PROGRAM IOMapping
VAR
	GasAnalogRead	: ARRAY[250..269] OF AnalogConverter ;
	ExhAnalogRead	: ARRAY[300..335] OF AnalogConverter ;
	OpAnalogRead	: ARRAY[600..607] OF AnalogConverter ;
	AV				: ARRAY[1..250] OF Valve ;
	bEMOStatus		: BOOL;
	aForceOpValve	: ARRAY[1..250] OF BOOL;
	AV65Open: Valve;
	bForceAV65Open: BOOL;
	AV65Close: Valve;
	bForceAV65Close: BOOL;
	AV202Open: Valve;
	AV202Close:Valve ;
	bForceAV202Open: BOOL;
	bForceAV202Close: BOOL;
	AV79Open: Valve;
	bForceAV79Open: BOOL;
	bForceAV79Close: BOOL;
	AV79Close: Valve;
	rO2Range: REAL;
	AV91Open: Valve;
	bForceAV91Open: BOOL;
	AV91Close: Valve;
	bForceAV91Close: BOOL;
END_VAR

Input();
Output();
Analog();
ValveCtrl();
ValveMapping();
PLC_to_PMC();
PMC_to_PLC();

ACTION Analog:
//模拟量读值转换实际读值程序
GasAnalogRead[250](	// PG/PS3 NH3 in pipe pressure
	AnalogRdValue_In_Int:= stGBI.IW250 , 
	AnalogResMin_In_Int:= 0 , 
	AnalogResMax_In_Int:= 32767 , 
	AnalogPhyMin_In_Real:= -0.1 , 
	AnalogPhyMax_In_Real:= 1 , 
	AnalogRdOffset_In_Real:= , 
	ActRdValue_Out_Real=> GVL.stPLCtoPMC.PG3_Pressure );
	
GasAnalogRead[251](	// PG/PS4 NH3-2 in pipe pressure
	AnalogRdValue_In_Int:= stGBI.IW251 , 
	AnalogResMin_In_Int:= 0 , 
	AnalogResMax_In_Int:= 32767 , 
	AnalogPhyMin_In_Real:= -0.1 , 
	AnalogPhyMax_In_Real:= 1 , 
	AnalogRdOffset_In_Real:= , 
	ActRdValue_Out_Real=> GVL.stPLCtoPMC.PG4_Pressure );

GasAnalogRead[252](	// PG/PS5 SiH4 in pipe pressure
	AnalogRdValue_In_Int:= stGBI.IW252 , 
	AnalogResMin_In_Int:= 0 , 
	AnalogResMax_In_Int:= 32767 , 
	AnalogPhyMin_In_Real:= -0.1 , 
	AnalogPhyMax_In_Real:= 1 , 
	AnalogRdOffset_In_Real:= , 
	ActRdValue_Out_Real=> GVL.stPLCtoPMC.PG5_Pressure );

GasAnalogRead[253](	// PG/PS6 N2-2 in pipe pressure
	AnalogRdValue_In_Int:= stGBI.IW253 , 
	AnalogResMin_In_Int:= 0 , 
	AnalogResMax_In_Int:= 32767 , 
	AnalogPhyMin_In_Real:= -0.1 , 
	AnalogPhyMax_In_Real:= 1 , 
	AnalogRdOffset_In_Real:= , 
	ActRdValue_Out_Real=> GVL.stPLCtoPMC.PG6_Pressure );
	
GasAnalogRead[254](	// PG/PS7 NF3 in pipe pressure
	AnalogRdValue_In_Int:= stGBI.IW254 , 
	AnalogResMin_In_Int:= 0 , 
	AnalogResMax_In_Int:= 32767 , 
	AnalogPhyMin_In_Real:= -0.1 , 
	AnalogPhyMax_In_Real:= 1 , 
	AnalogRdOffset_In_Real:= , 
	ActRdValue_Out_Real=> GVL.stPLCtoPMC.PG7_Pressure );
	
GasAnalogRead[255](	// PG/PS8 20%F2/N2 in pipe pressure
	AnalogRdValue_In_Int:= stGBI.IW255 ,  
	AnalogResMin_In_Int:= 0 , 
	AnalogResMax_In_Int:= 32767 , 
	AnalogPhyMin_In_Real:= -0.1 , 
	AnalogPhyMax_In_Real:= 1 , 
	AnalogRdOffset_In_Real:= , 
	ActRdValue_Out_Real=> GVL.stPLCtoPMC.PG8_Pressure );
	
GasAnalogRead[256](	// PG/PS31 N2-10 in pipe pressure
	AnalogRdValue_In_Int:= stGBI.IW256 , 
	AnalogResMin_In_Int:= 0 , 
	AnalogResMax_In_Int:= 32767 , 
	AnalogPhyMin_In_Real:= -0.1 , 
	AnalogPhyMax_In_Real:= 1 , 
	AnalogRdOffset_In_Real:= , 
	ActRdValue_Out_Real=> GVL.stPLCtoPMC.PG31_Pressure );
	
GasAnalogRead[257](	// PG/PS32 N2-11 in pipe pressure
	AnalogRdValue_In_Int:= stGBI.IW257 , 
	AnalogResMin_In_Int:= 0 , 
	AnalogResMax_In_Int:= 32767 , 
	AnalogPhyMin_In_Real:= -0.1 , 
	AnalogPhyMax_In_Real:= 1 , 
	AnalogRdOffset_In_Real:= , 
	ActRdValue_Out_Real=> GVL.stPLCtoPMC.PG32_Pressure );
	
GasAnalogRead[258](	// VG31 tank-1 backward pipe pressure (0~100torr)
	AnalogRdValue_In_Int:= stGBI.IW258 , 
	AnalogResMin_In_Int:= 0 , 
	AnalogResMax_In_Int:= 32767 , 
	AnalogPhyMin_In_Real:= 0 , 
	AnalogPhyMax_In_Real:= 100 , 
	AnalogRdOffset_In_Real:= , 
	ActRdValue_Out_Real=> GVL.stPLCtoPMC.VG31_Pressure );
	
GasAnalogRead[259](	// PG/PS2 HCL pressure
	AnalogRdValue_In_Int:= stGBI.IW259 , 
	AnalogResMin_In_Int:= 0 , 
	AnalogResMax_In_Int:= 32767 , 
	AnalogPhyMin_In_Real:= -0.1 , 
	AnalogPhyMax_In_Real:= 1 , 
	AnalogRdOffset_In_Real:= , 
	ActRdValue_Out_Real=> GVL.stPLCtoPMC.OX_Value );
	
GasAnalogRead[260](	// PS11 N2-8 in pipe pressure
	AnalogRdValue_In_Int:= stGBI.IW260 , 
	AnalogResMin_In_Int:= 1996 , 
	AnalogResMax_In_Int:= 16383 , 
	AnalogPhyMin_In_Real:= 0 , 
	AnalogPhyMax_In_Real:= 1 , 
	AnalogRdOffset_In_Real:= , 
	ActRdValue_Out_Real=> GVL.stPLCtoPMC.PS11_Pressure );
	
GasAnalogRead[261](	// PG/PS1 N2-1 in pipe pressure
	AnalogRdValue_In_Int:= stGBI.IW261 , 
	AnalogResMin_In_Int:= 0 , 
	AnalogResMax_In_Int:= 32767 , 
	AnalogPhyMin_In_Real:= -0.1 , 
	AnalogPhyMax_In_Real:= 1 , 
	AnalogRdOffset_In_Real:= , 
	ActRdValue_Out_Real=> GVL.stPLCtoPMC.PG1_Pressure );
	
GasAnalogRead[262](	// MS2 gas box(左) exhaust pressure
	AnalogRdValue_In_Int:= stGBI.IW262 , 
	AnalogResMin_In_Int:= 0 , 
	AnalogResMax_In_Int:= 32767 , 
	AnalogPhyMin_In_Real:= 0 , 
	AnalogPhyMax_In_Real:= 200 , 
	AnalogRdOffset_In_Real:= , 
	ActRdValue_Out_Real=> GVL.stPLCtoPMC.MS2_Gasboxleft );
	
GasAnalogRead[263]( // MS5 loading area exhaust pressure
	AnalogRdValue_In_Int:= stGBI.IW263 , 
	AnalogResMin_In_Int:= 0 , 
	AnalogResMax_In_Int:= 32767 , 
	AnalogPhyMin_In_Real:= 0 , 
	AnalogPhyMax_In_Real:= 200 , 
	AnalogRdOffset_In_Real:= , 
	ActRdValue_Out_Real=> GVL.stPLCtoPMC.MS5_Loadingarea );
	

//O2 Range judgment
IF NOT stGBI.I201_13 AND stGBI.I201_14 AND stGBI.I201_15 THEN
	rO2Range := 1000000 ; // O2 range 0~100%
END_IF

IF stGBI.I201_13 AND NOT stGBI.I201_14 AND stGBI.I201_15 THEN
	rO2Range := 100000 ; // O2 range 0~10%
END_IF

IF NOT stGBI.I201_13 AND NOT stGBI.I201_14 AND stGBI.I201_15 THEN
	rO2Range := 10000 ; // O2 range 0~1%
END_IF

IF stGBI.I201_13 AND stGBI.I201_14 AND NOT stGBI.I201_15 THEN
	rO2Range := 1000 ; // O2 range 0~1000ppm
END_IF

IF NOT stGBI.I201_13 AND stGBI.I201_14 AND NOT stGBI.I201_15 THEN
	rO2Range := 100 ; // O2 range 0~100ppm
END_IF

IF stGBI.I201_13 AND NOT stGBI.I201_14 AND NOT stGBI.I201_15 THEN
	rO2Range := 10 ; // O2 range 0~10ppm
END_IF

GasAnalogRead[264](	// O2 concention
	AnalogRdValue_In_Int:= stGBI.IW264 ,  
	AnalogResMin_In_Int:= 0 , 
	AnalogResMax_In_Int:= 32767 , 
	AnalogPhyMin_In_Real:= 0 , 
	AnalogPhyMax_In_Real:= rO2Range , 
	AnalogRdOffset_In_Real:= , 
	ActRdValue_Out_Real=> GVL.stPLCtoPMC.OX_Value );
	
GasAnalogRead[265](	// spare
	AnalogRdValue_In_Int:= stGBI.IW265 , 
	AnalogResMin_In_Int:= 0 , 
	AnalogResMax_In_Int:= 32767 , 
	AnalogPhyMin_In_Real:= 0 , 
	AnalogPhyMax_In_Real:= 1 , 
	AnalogRdOffset_In_Real:= , 
	ActRdValue_Out_Real=> );
	
GasAnalogRead[266](	// PG/PS21 Tank-1 forward pipe pressure
	AnalogRdValue_In_Int:= stGBI.IW266 , 
	AnalogResMin_In_Int:= 3277 , 
	AnalogResMax_In_Int:= 16383 , 
	AnalogPhyMin_In_Real:= -100 , 
	AnalogPhyMax_In_Real:= 300 , 
	AnalogRdOffset_In_Real:= , 
	ActRdValue_Out_Real=> GVL.stPLCtoPMC.PG21_Pressure );
	
GasAnalogRead[267](	// PG/PS22 Tank-2 forward pipe pressure
	AnalogRdValue_In_Int:= stGBI.IW267 , 
	AnalogResMin_In_Int:= 3277 , 
	AnalogResMax_In_Int:= 16383 , 
	AnalogPhyMin_In_Real:= -100 , 
	AnalogPhyMax_In_Real:= 300 , 
	AnalogRdOffset_In_Real:= , 
	ActRdValue_Out_Real=> GVL.stPLCtoPMC.PG22_Pressure );
	
GasAnalogRead[268](	// PG/PS23 Tank-3 forward pipe pressure
	AnalogRdValue_In_Int:= stGBI.IW268 , 
	AnalogResMin_In_Int:= 3277 , 
	AnalogResMax_In_Int:= 16383 , 
	AnalogPhyMin_In_Real:= -100 , 
	AnalogPhyMax_In_Real:= 300 , 
	AnalogRdOffset_In_Real:= , 
	ActRdValue_Out_Real=> GVL.stPLCtoPMC.PG23_Pressure );
	
GasAnalogRead[269](	// PS33  LSC tank pressure
	AnalogRdValue_In_Int:= stGBI.IW269 ,  
	AnalogResMin_In_Int:= 3277 , 
	AnalogResMax_In_Int:= 16383 , 
	AnalogPhyMin_In_Real:= -100 , 
	AnalogPhyMax_In_Real:= 500 , 
	AnalogRdOffset_In_Real:= , 
	ActRdValue_Out_Real=> GVL.stPLCtoPMC.PS33_Pressure );	
	
ExhAnalogRead[300](	// FS105 RHC cooling water flow
	AnalogRdValue_In_Int:= stEXHI.IW300 , 
	AnalogResMin_In_Int:= 0 ,
	AnalogResMax_In_Int:= 32767 , 
	AnalogPhyMin_In_Real:= 0 , 
	AnalogPhyMax_In_Real:= 40 , 
	AnalogRdOffset_In_Real:= , 
	ActRdValue_Out_Real=> GVL.stPLCtoPMC.FS105_Flow );
	
ExhAnalogRead[301](	// FS106 Heater jacket cooling water flow
	AnalogRdValue_In_Int:= stEXHI.IW301 , 
	AnalogResMin_In_Int:= 0 ,
	AnalogResMax_In_Int:= 32767 , 
	AnalogPhyMin_In_Real:= 0 , 
	AnalogPhyMax_In_Real:= 16 , 
	AnalogRdOffset_In_Real:= , 
	ActRdValue_Out_Real=> GVL.stPLCtoPMC.FS106_Flow );
	
ExhAnalogRead[302](	// FS202 Furnace cooling water flow
	AnalogRdValue_In_Int:= stEXHI.IW302 , 
	AnalogResMin_In_Int:= 0 ,
	AnalogResMax_In_Int:= 32767 , 
	AnalogPhyMin_In_Real:= 0 , 
	AnalogPhyMax_In_Real:= 16 , 
	AnalogRdOffset_In_Real:= , 
	ActRdValue_Out_Real=> GVL.stPLCtoPMC.FS202_Flow );
	
ExhAnalogRead[303](	// FS104 Shutter cooling water flow
	AnalogRdValue_In_Int:= stEXHI.IW303 , 
	AnalogResMin_In_Int:= 0 ,
	AnalogResMax_In_Int:= 32767 , 
	AnalogPhyMin_In_Real:= 0 , 
	AnalogPhyMax_In_Real:= 4 , 
	AnalogRdOffset_In_Real:= , 
	ActRdValue_Out_Real=> GVL.stPLCtoPMC.FS104_Flow );
	
ExhAnalogRead[304](	// FS111 boat rotation cooling water flow
	AnalogRdValue_In_Int:= stEXHI.IW304 , 
	AnalogResMin_In_Int:= 0 ,
	AnalogResMax_In_Int:= 32767 , 
	AnalogPhyMin_In_Real:= 0 , 
	AnalogPhyMax_In_Real:= 4 , 
	AnalogRdOffset_In_Real:= , 
	ActRdValue_Out_Real=> GVL.stPLCtoPMC.FS111_Flow );
	
ExhAnalogRead[305](	// FS102 Flange cooling water flow
	AnalogRdValue_In_Int:= stEXHI.IW305 , 
	AnalogResMin_In_Int:= 0 ,
	AnalogResMax_In_Int:= 32767 , 
	AnalogPhyMin_In_Real:= 0 , 
	AnalogPhyMax_In_Real:= 4 , 
	AnalogRdOffset_In_Real:= , 
	ActRdValue_Out_Real=> GVL.stPLCtoPMC.FS102_Flow );
	
ExhAnalogRead[306](	// spare
	AnalogRdValue_In_Int:= stEXHI.IW306 , 
	AnalogResMin_In_Int:= 0 ,
	AnalogResMax_In_Int:= 32767 , 
	AnalogPhyMin_In_Real:= 0 , 
	AnalogPhyMax_In_Real:= 1 , 
	AnalogRdOffset_In_Real:= , 
	ActRdValue_Out_Real=> );
	
ExhAnalogRead[307](	// spare
	AnalogRdValue_In_Int:= stEXHI.IW307 , 
	AnalogResMin_In_Int:= 0 ,
	AnalogResMax_In_Int:= 32767 , 
	AnalogPhyMin_In_Real:= 0 , 
	AnalogPhyMax_In_Real:= 1 , 
	AnalogRdOffset_In_Real:= , 
	ActRdValue_Out_Real=> );
	
ExhAnalogRead[308](	// DG1 tube and loading area differential pressure
	AnalogRdValue_In_Int:= stEXHI.IW308 , 
	AnalogResMin_In_Int:= 0 ,
	AnalogResMax_In_Int:= 32767 , 
	AnalogPhyMin_In_Real:= -300 , 
	AnalogPhyMax_In_Real:= 300 , 
	AnalogRdOffset_In_Real:= , 
	ActRdValue_Out_Real=> GVL.stPLCtoPMC.DG1_Pressure );
	
ExhAnalogRead[309](	// spare
	AnalogRdValue_In_Int:= stEXHI.IW309 , 
	AnalogResMin_In_Int:= 0 ,
	AnalogResMax_In_Int:= 32767 , 
	AnalogPhyMin_In_Real:= 0 , 
	AnalogPhyMax_In_Real:= 1 , 
	AnalogRdOffset_In_Real:= , 
	ActRdValue_Out_Real=> );
	
ExhAnalogRead[310](	// spare
	AnalogRdValue_In_Int:= stEXHI.IW310 , 
	AnalogResMin_In_Int:= 0 ,
	AnalogResMax_In_Int:= 32767 , 
	AnalogPhyMin_In_Real:= 0 , 
	AnalogPhyMax_In_Real:= 1 , 
	AnalogRdOffset_In_Real:= , 
	ActRdValue_Out_Real=> );
	
ExhAnalogRead[311](	// FS116 Cooling unit flow
	AnalogRdValue_In_Int:= stEXHI.IW311 , 
	AnalogResMin_In_Int:= 0 ,
	AnalogResMax_In_Int:= 32767 , 
	AnalogPhyMin_In_Real:= 0 , 
	AnalogPhyMax_In_Real:= 16 , 
	AnalogRdOffset_In_Real:= , 
	ActRdValue_Out_Real=> GVL.stPLCtoPMC.FS116_Flow );
	
ExhAnalogRead[312](	// PS13 pressure
	AnalogRdValue_In_Int:= stEXHI.IW312 , 
	AnalogResMin_In_Int:= 0 ,
	AnalogResMax_In_Int:= 32767 , 
	AnalogPhyMin_In_Real:= 0 , 
	AnalogPhyMax_In_Real:= 98.1 , 
	AnalogRdOffset_In_Real:= , 
	ActRdValue_Out_Real=> GVL.stPLCtoPMC.PS13_Pressure );
	
ExhAnalogRead[313](	// spare
	AnalogRdValue_In_Int:= stEXHI.IW313 , 
	AnalogResMin_In_Int:= 0 ,
	AnalogResMax_In_Int:= 32767 , 
	AnalogPhyMin_In_Real:= 0 , 
	AnalogPhyMax_In_Real:= 1 , 
	AnalogRdOffset_In_Real:= , 
	ActRdValue_Out_Real=> );
	
ExhAnalogRead[314](	// spare
	AnalogRdValue_In_Int:= stEXHI.IW314 , 
	AnalogResMin_In_Int:= 0 ,
	AnalogResMax_In_Int:= 32767 , 
	AnalogPhyMin_In_Real:= 0 , 
	AnalogPhyMax_In_Real:= 1 , 
	AnalogRdOffset_In_Real:= , 
	ActRdValue_Out_Real=> );
	
ExhAnalogRead[315](	// spare
	AnalogRdValue_In_Int:= stEXHI.IW315 , 
	AnalogResMin_In_Int:= 0 ,
	AnalogResMax_In_Int:= 32767 , 
	AnalogPhyMin_In_Real:= 0 , 
	AnalogPhyMax_In_Real:= 1 , 
	AnalogRdOffset_In_Real:= , 
	ActRdValue_Out_Real=> );
	
ExhAnalogRead[316](	// spare
	AnalogRdValue_In_Int:= stEXHI.IW316 , 
	AnalogResMin_In_Int:= 0 ,
	AnalogResMax_In_Int:= 32767 , 
	AnalogPhyMin_In_Real:= 0 , 
	AnalogPhyMax_In_Real:= 1 , 
	AnalogRdOffset_In_Real:= , 
	ActRdValue_Out_Real=> );
	
ExhAnalogRead[317](	// spare
	AnalogRdValue_In_Int:= stEXHI.IW317 , 
	AnalogResMin_In_Int:= 0 ,
	AnalogResMax_In_Int:= 32767 , 
	AnalogPhyMin_In_Real:= 0 , 
	AnalogPhyMax_In_Real:= 1 , 
	AnalogRdOffset_In_Real:= , 
	ActRdValue_Out_Real=> );
	
ExhAnalogRead[318](	// PS21 N2-13 in pipe pressure 0.6~5V
	AnalogRdValue_In_Int:= stEXHI.IW318 , 
	AnalogResMin_In_Int:= 3276 ,
	AnalogResMax_In_Int:= 16383 , 
	AnalogPhyMin_In_Real:= -0.1 , 
	AnalogPhyMax_In_Real:= 1 , 
	AnalogRdOffset_In_Real:= , 
	ActRdValue_Out_Real=> GVL.stPLCtoPMC.PS21_Pressure );
	
ExhAnalogRead[319](	// PS110 exhaust pressure
	AnalogRdValue_In_Int:= stEXHI.IW319 , 
	AnalogResMin_In_Int:= 3276 ,
	AnalogResMax_In_Int:= 16383 , 
	AnalogPhyMin_In_Real:= -100 , 
	AnalogPhyMax_In_Real:= 100 , 
	AnalogRdOffset_In_Real:= , 
	ActRdValue_Out_Real=> GVL.stPLCtoPMC.PS110_Pressure );
	
ExhAnalogRead[320](	// PG/PS12 N2-9 in pipe pressure
	AnalogRdValue_In_Int:= stEXHI.IW320 , 
	AnalogResMin_In_Int:= 0 ,
	AnalogResMax_In_Int:= 32767 , 
	AnalogPhyMin_In_Real:= -0.1 , 
	AnalogPhyMax_In_Real:= 1 , 
	AnalogRdOffset_In_Real:= , 
	ActRdValue_Out_Real=> GVL.stPLCtoPMC.PG12_Pressure );
	
ExhAnalogRead[321](	// VG14 pressure
	AnalogRdValue_In_Int:= stEXHI.IW321 , 
	AnalogResMin_In_Int:= 0 ,
	AnalogResMax_In_Int:= 32767 , 
	AnalogPhyMin_In_Real:= 0 , 
	AnalogPhyMax_In_Real:= 10 , 
	AnalogRdOffset_In_Real:= , 
	ActRdValue_Out_Real=> GVL.stPLCtoPMC.VG14_Pressure );
	
ExhAnalogRead[322](	// PS14 pressure
	AnalogRdValue_In_Int:= stEXHI.IW322 , 
	AnalogResMin_In_Int:= 3276 ,
	AnalogResMax_In_Int:= 16383 , 
	AnalogPhyMin_In_Real:= -100 , 
	AnalogPhyMax_In_Real:= 100 , 
	AnalogRdOffset_In_Real:= , 
	ActRdValue_Out_Real=> GVL.stPLCtoPMC.PS14_Pressure );
	
ExhAnalogRead[323](	// spare
	AnalogRdValue_In_Int:= stEXHI.IW323 , 
	AnalogResMin_In_Int:= 0 ,
	AnalogResMax_In_Int:= 32767 , 
	AnalogPhyMin_In_Real:= 0 , 
	AnalogPhyMax_In_Real:= 1 , 
	AnalogRdOffset_In_Real:= , 
	ActRdValue_Out_Real=> );
	
ExhAnalogRead[324](	// spare
	AnalogRdValue_In_Int:= stEXHI.IW324 , 
	AnalogResMin_In_Int:= 0 ,
	AnalogResMax_In_Int:= 32767 , 
	AnalogPhyMin_In_Real:= 0 , 
	AnalogPhyMax_In_Real:= 1 , 
	AnalogRdOffset_In_Real:= , 
	ActRdValue_Out_Real=> );
	
ExhAnalogRead[325](	// spare
	AnalogRdValue_In_Int:= stEXHI.IW325 , 
	AnalogResMin_In_Int:= 0 ,
	AnalogResMax_In_Int:= 32767 , 
	AnalogPhyMin_In_Real:= 0 , 
	AnalogPhyMax_In_Real:= 1 , 
	AnalogRdOffset_In_Real:= , 
	ActRdValue_Out_Real=> );
	
ExhAnalogRead[326](	// spare
	AnalogRdValue_In_Int:= stEXHI.IW326 , 
	AnalogResMin_In_Int:= 0 ,
	AnalogResMax_In_Int:= 32767 , 
	AnalogPhyMin_In_Real:= 0 , 
	AnalogPhyMax_In_Real:= 1 , 
	AnalogRdOffset_In_Real:= , 
	ActRdValue_Out_Real=> );
	
ExhAnalogRead[327](	// spare
	AnalogRdValue_In_Int:= stEXHI.IW327 , 
	AnalogResMin_In_Int:= 0 ,
	AnalogResMax_In_Int:= 32767 , 
	AnalogPhyMin_In_Real:= 0 , 
	AnalogPhyMax_In_Real:= 1 , 
	AnalogRdOffset_In_Real:= , 
	ActRdValue_Out_Real=> );
	
ExhAnalogRead[328](	// spare
	AnalogRdValue_In_Int:= stEXHI.IW328 , 
	AnalogResMin_In_Int:= 0 ,
	AnalogResMax_In_Int:= 32767 , 
	AnalogPhyMin_In_Real:= 0 , 
	AnalogPhyMax_In_Real:= 1 , 
	AnalogRdOffset_In_Real:= , 
	ActRdValue_Out_Real=> );
	
ExhAnalogRead[329](	// spare
	AnalogRdValue_In_Int:= stEXHI.IW329 , 
	AnalogResMin_In_Int:= 0 ,
	AnalogResMax_In_Int:= 32767 , 
	AnalogPhyMin_In_Real:= 0 , 
	AnalogPhyMax_In_Real:= 1 , 
	AnalogRdOffset_In_Real:= , 
	ActRdValue_Out_Real=> );
	
ExhAnalogRead[330](	// spare
	AnalogRdValue_In_Int:= stEXHI.IW330 , 
	AnalogResMin_In_Int:= 0 ,
	AnalogResMax_In_Int:= 32767 , 
	AnalogPhyMin_In_Real:= 0 , 
	AnalogPhyMax_In_Real:= 1 , 
	AnalogRdOffset_In_Real:= , 
	ActRdValue_Out_Real=> );
	
ExhAnalogRead[331](	// spare
	AnalogRdValue_In_Int:= stEXHI.IW331 , 
	AnalogResMin_In_Int:= 0 ,
	AnalogResMax_In_Int:= 32767 , 
	AnalogPhyMin_In_Real:= 0 , 
	AnalogPhyMax_In_Real:= 1 , 
	AnalogRdOffset_In_Real:= , 
	ActRdValue_Out_Real=> );
	
ExhAnalogRead[332](	// spare
	AnalogRdValue_In_Int:= stEXHI.IW332 , 
	AnalogResMin_In_Int:= 0 ,
	AnalogResMax_In_Int:= 32767 , 
	AnalogPhyMin_In_Real:= 0 , 
	AnalogPhyMax_In_Real:= 1 , 
	AnalogRdOffset_In_Real:= , 
	ActRdValue_Out_Real=> );
	
ExhAnalogRead[333](	// spare
	AnalogRdValue_In_Int:= stEXHI.IW333 , 
	AnalogResMin_In_Int:= 0 ,
	AnalogResMax_In_Int:= 32767 , 
	AnalogPhyMin_In_Real:= 0 , 
	AnalogPhyMax_In_Real:= 1 , 
	AnalogRdOffset_In_Real:= , 
	ActRdValue_Out_Real=> );
	
ExhAnalogRead[334](	// spare
	AnalogRdValue_In_Int:= stEXHI.IW334 , 
	AnalogResMin_In_Int:= 0 ,
	AnalogResMax_In_Int:= 32767 , 
	AnalogPhyMin_In_Real:= 0 , 
	AnalogPhyMax_In_Real:= 1 , 
	AnalogRdOffset_In_Real:= , 
	ActRdValue_Out_Real=> );
	
ExhAnalogRead[335](	// spare
	AnalogRdValue_In_Int:= stEXHI.IW335 , 
	AnalogResMin_In_Int:= 0 ,
	AnalogResMax_In_Int:= 32767 , 
	AnalogPhyMin_In_Real:= 0 , 
	AnalogPhyMax_In_Real:= 1 , 
	AnalogRdOffset_In_Real:= , 
	ActRdValue_Out_Real=> );
	
OpAnalogRead[600](	// MS8 RHC exhaust pressure
	AnalogRdValue_In_Int:= stOPI.IW600 , 
	AnalogResMin_In_Int:= 0 ,
	AnalogResMax_In_Int:= 32767 , 
	AnalogPhyMin_In_Real:= 0 , 
	AnalogPhyMax_In_Real:= 2 , 
	AnalogRdOffset_In_Real:= , 
	ActRdValue_Out_Real=> GVL.stPLCtoPMC.MS8_RHC_ExhPress );
	
OpAnalogRead[601](	// MS1 Heater exhaust pressure
	AnalogRdValue_In_Int:= stOPI.IW601 , 
	AnalogResMin_In_Int:= 0 ,
	AnalogResMax_In_Int:= 32767 , 
	AnalogPhyMin_In_Real:= 0 , 
	AnalogPhyMax_In_Real:= 200 , 
	AnalogRdOffset_In_Real:= , 
	ActRdValue_Out_Real=> GVL.stPLCtoPMC.MS1_Heater );
	
OpAnalogRead[602](	// MS3 Scavenger exhaust pressure
	AnalogRdValue_In_Int:= stOPI.IW602 , 
	AnalogResMin_In_Int:= 0 ,
	AnalogResMax_In_Int:= 32767 , 
	AnalogPhyMin_In_Real:= 0 , 
	AnalogPhyMax_In_Real:= 200 , 
	AnalogRdOffset_In_Real:= , 
	ActRdValue_Out_Real=> GVL.stPLCtoPMC.MS3_Scavenger );
	
OpAnalogRead[603](	// MS6 Frontbody exhaust pressure
	AnalogRdValue_In_Int:= stOPI.IW603 , 
	AnalogResMin_In_Int:= 0 ,
	AnalogResMax_In_Int:= 32767 , 
	AnalogPhyMin_In_Real:= 0 , 
	AnalogPhyMax_In_Real:= 200 , 
	AnalogRdOffset_In_Real:= , 
	ActRdValue_Out_Real=> GVL.stPLCtoPMC.MS6_Frontbody );
	
OpAnalogRead[604](	// MS9 LSC1 exhaust pressure
	AnalogRdValue_In_Int:= stOPI.IW604 , 
	AnalogResMin_In_Int:= 0 ,
	AnalogResMax_In_Int:= 32767 , 
	AnalogPhyMin_In_Real:= 0 , 
	AnalogPhyMax_In_Real:= 200 , 
	AnalogRdOffset_In_Real:= , 
	ActRdValue_Out_Real=> GVL.stPLCtoPMC.MS9_LSC1 );
	
OpAnalogRead[605](	// MS11 Gas box(右上) exhaust pressure
	AnalogRdValue_In_Int:= stOPI.IW605 , 
	AnalogResMin_In_Int:= 0 ,
	AnalogResMax_In_Int:= 32767 , 
	AnalogPhyMin_In_Real:= 0 , 
	AnalogPhyMax_In_Real:= 200 , 
	AnalogRdOffset_In_Real:= , 
	ActRdValue_Out_Real=> GVL.stPLCtoPMC.MS11_GasBox );
	
OpAnalogRead[606](	// MS12 Gas box(右下) exhaust pressure
	AnalogRdValue_In_Int:= stOPI.IW606 , 
	AnalogResMin_In_Int:= 0 ,
	AnalogResMax_In_Int:= 32767 , 
	AnalogPhyMin_In_Real:= 0 , 
	AnalogPhyMax_In_Real:= 200 , 
	AnalogRdOffset_In_Real:= , 
	ActRdValue_Out_Real=> GVL.stPLCtoPMC.MS12_GasBox );
	
OpAnalogRead[607](	// spare
	AnalogRdValue_In_Int:= stOPI.IW607 , 
	AnalogResMin_In_Int:= 0 ,
	AnalogResMax_In_Int:= 32767 , 
	AnalogPhyMin_In_Real:= 0 , 
	AnalogPhyMax_In_Real:= 200 , 
	AnalogRdOffset_In_Real:= , 
	ActRdValue_Out_Real=> );
END_ACTION

ACTION Input:
//************************************************************************
//02.Gas Box INput/OUTPUT(气体柜输入/出映射）
//************************************************************************
stGBI.	I200_00	:=		GB_EL1889[1,0]	;
stGBI.	I200_01	:=		GB_EL1889[1,1]	;
stGBI.	I200_02	:=		GB_EL1889[1,2]	;
stGBI.	I200_03	:=		GB_EL1889[1,3]	;
stGBI.	I200_04	:=		GB_EL1889[1,4]	;
stGBI.	I200_05	:=		GB_EL1889[1,5]	;
stGBI.	I200_06	:=		GB_EL1889[1,6]	;
stGBI.	I200_07	:=		GB_EL1889[1,7]	;
stGBI.	I200_08	:=		GB_EL1889[1,8]	;
stGBI.	I200_09	:=		GB_EL1889[1,9]	;
stGBI.	I200_10	:=		GB_EL1889[1,10]	;
stGBI.	I200_11	:=		GB_EL1889[1,11]	;
stGBI.	I200_12	:=		GB_EL1889[1,12]	;
stGBI.	I200_13	:=		GB_EL1889[1,13]	;
stGBI.	I200_14	:=		GB_EL1889[1,14]	;
stGBI.	I200_15	:=		GB_EL1889[1,15]	;
stGBI.	I201_00	:=		GB_EL1889[2,0]	;
stGBI.	I201_01	:=		GB_EL1889[2,1]	;
stGBI.	I201_02	:=		GB_EL1889[2,2]	;
stGBI.	I201_03	:=		GB_EL1889[2,3]	;
stGBI.	I201_04	:=		GB_EL1889[2,4]	;
stGBI.	I201_05	:=		GB_EL1889[2,5]	;
stGBI.	I201_06	:=		GB_EL1889[2,6]	;
stGBI.	I201_07	:=		GB_EL1889[2,7]	;
stGBI.	I201_08	:=		GB_EL1889[2,8]	;
stGBI.	I201_09	:=		GB_EL1889[2,9]	;
stGBI.	I201_10	:=		GB_EL1889[2,10]	;
stGBI.	I201_11	:=		GB_EL1889[2,11]	;
stGBI.	I201_12	:=		GB_EL1889[2,12]	;
stGBI.	I201_13	:=		GB_EL1889[2,13]	;
stGBI.	I201_14	:=		GB_EL1889[2,14]	;
stGBI.	I201_15	:=		GB_EL1889[2,15]	;
stGBI.	I203_00	:=		GB_EL1889[3,0]	;
stGBI.	I203_01	:=		GB_EL1889[3,1]	;
stGBI.	I203_02	:=		GB_EL1889[3,2]	;
stGBI.	I203_03	:=		GB_EL1889[3,3]	;
stGBI.	I203_04	:=		GB_EL1889[3,4]	;
stGBI.	I203_05	:=		GB_EL1889[3,5]	;
stGBI.	I203_06	:=		GB_EL1889[3,6]	;
stGBI.	I203_07	:=		GB_EL1889[3,7]	;
stGBI.	I203_08	:=		GB_EL1889[3,8]	;
stGBI.	I203_09	:=		GB_EL1889[3,9]	;
stGBI.	I203_10	:=		GB_EL1889[3,10]	;
stGBI.	I203_11	:=		GB_EL1889[3,11]	;
stGBI.	I203_12	:=		GB_EL1889[3,12]	;
stGBI.	I203_13	:=		GB_EL1889[3,13]	;
stGBI.	I203_14	:=		GB_EL1889[3,14]	;
stGBI.	I203_15	:=		GB_EL1889[3,15]	;

stGBI.	IW250	:=		GB_EL3164[1,	1]	;
stGBI.	IW251	:=		GB_EL3164[1,	2]	;
stGBI.	IW252	:=		GB_EL3164[1,	3]	;
stGBI.	IW253	:=		GB_EL3164[1,	4]	;
stGBI.	IW254	:=		GB_EL3164[2,	1]	;
stGBI.	IW255	:=		GB_EL3164[2,	2]	;
stGBI.	IW256	:=		GB_EL3164[2,	3]	;
stGBI.	IW257	:=		GB_EL3164[2,	4]	;
stGBI.	IW258	:=		GB_EL3164[3,	1]	;
stGBI.	IW259	:=		GB_EL3164[3,	2]	;
stGBI.	IW260	:=		GB_EL3164[3,	3]	;
stGBI.	IW261	:=		GB_EL3164[3,	4]	;
stGBI.	IW262	:=		GB_EL3124[1,	1]	;
stGBI.	IW263	:=		GB_EL3124[1,	2]	;
stGBI.	IW264	:=		GB_EL3124[1,	3]	;
stGBI.	IW265	:=		GB_EL3124[1,	4]	;
stGBI.	IW266	:=		GB_EL3164[4,	1]	;
stGBI.	IW267	:=		GB_EL3164[4,	2]	;
stGBI.	IW268	:=		GB_EL3164[4,	3]	;
stGBI.	IW269	:=		GB_EL3164[4,	4]	;


//************************************************************************
//03.EXH Box INput/OUTPUT(排气柜输入/出映射）
//************************************************************************
stEXHI.	I300_00	:=		EXH_EL1889[1,0]	;
stEXHI.	I300_01	:=		EXH_EL1889[1,1]	;
stEXHI.	I300_02	:=		EXH_EL1889[1,2]	;
stEXHI.	I300_03	:=		EXH_EL1889[1,3]	;
stEXHI.	I300_04	:=		EXH_EL1889[1,4]	;
stEXHI.	I300_05	:=		EXH_EL1889[1,5]	;
stEXHI.	I300_06	:=		EXH_EL1889[1,6]	;
stEXHI.	I300_07	:=		EXH_EL1889[1,7]	;
stEXHI.	I300_08	:=		EXH_EL1889[1,8]	;
stEXHI.	I300_09	:=		EXH_EL1889[1,9]	;
stEXHI.	I300_10	:=		EXH_EL1889[1,10]	;
stEXHI.	I300_11	:=		EXH_EL1889[1,11]	;
stEXHI.	I300_12	:=		EXH_EL1889[1,12]	;
stEXHI.	I300_13	:=		EXH_EL1889[1,13]	;
stEXHI.	I300_14	:=		EXH_EL1889[1,14]	;
stEXHI.	I300_15	:=		EXH_EL1889[1,15]	;
stEXHI.	I301_00	:=		EXH_EL1889[2,0]	;
stEXHI.	I301_01	:=		EXH_EL1889[2,1]	;
stEXHI.	I301_02	:=		EXH_EL1889[2,2]	;
stEXHI.	I301_03	:=		EXH_EL1889[2,3]	;
stEXHI.	I301_04	:=		EXH_EL1889[2,4]	;
stEXHI.	I301_05	:=		EXH_EL1889[2,5]	;
stEXHI.	I301_06	:=		EXH_EL1889[2,6]	;
stEXHI.	I301_07	:=		EXH_EL1889[2,7]	;
stEXHI.	I301_08	:=		EXH_EL1889[2,8]	;
stEXHI.	I301_09	:=		EXH_EL1889[2,9]	;
stEXHI.	I301_10	:=		EXH_EL1889[2,10]	;
stEXHI.	I301_11	:=		EXH_EL1889[2,11]	;
stEXHI.	I301_12	:=		EXH_EL1889[2,12]	;
stEXHI.	I301_13	:=		EXH_EL1889[2,13]	;
stEXHI.	I301_14	:=		EXH_EL1889[2,14]	;
stEXHI.	I301_15	:=		EXH_EL1889[2,15]	;
stEXHI.	I302_00	:=		EXH_EL1889[3,0]	;
stEXHI.	I302_01	:=		EXH_EL1889[3,1]	;
stEXHI.	I302_02	:=		EXH_EL1889[3,2]	;
stEXHI.	I302_03	:=		EXH_EL1889[3,3]	;
stEXHI.	I302_04	:=		EXH_EL1889[3,4]	;
stEXHI.	I302_05	:=		EXH_EL1889[3,5]	;
stEXHI.	I302_06	:=		EXH_EL1889[3,6]	;
stEXHI.	I302_07	:=		EXH_EL1889[3,7]	;
stEXHI.	I302_08	:=		EXH_EL1889[3,8]	;
stEXHI.	I302_09	:=		EXH_EL1889[3,9]	;
stEXHI.	I302_10	:=		EXH_EL1889[3,10]	;
stEXHI.	I302_11	:=		EXH_EL1889[3,11]	;
stEXHI.	I302_12	:=		EXH_EL1889[3,12]	;
stEXHI.	I302_13	:=		EXH_EL1889[3,13]	;
stEXHI.	I302_14	:=		EXH_EL1889[3,14]	;
stEXHI.	I302_15	:=		EXH_EL1889[3,15]	;
stEXHI.	I303_00	:=		EXH_EL1889[4,0]	;
stEXHI.	I303_01	:=		EXH_EL1889[4,1]	;
stEXHI.	I303_02	:=		EXH_EL1889[4,2]	;
stEXHI.	I303_03	:=		EXH_EL1889[4,3]	;
stEXHI.	I303_04	:=		EXH_EL1889[4,4]	;
stEXHI.	I303_05	:=		EXH_EL1889[4,5]	;
stEXHI.	I303_06	:=		EXH_EL1889[4,6]	;
stEXHI.	I303_07	:=		EXH_EL1889[4,7]	;
stEXHI.	I303_08	:=		EXH_EL1889[4,8]	;
stEXHI.	I303_09	:=		EXH_EL1889[4,9]	;
stEXHI.	I303_10	:=		EXH_EL1889[4,10]	;
stEXHI.	I303_11	:=		EXH_EL1889[4,11]	;
stEXHI.	I303_12	:=		EXH_EL1889[4,12]	;
stEXHI.	I303_13	:=		EXH_EL1889[4,13]	;
stEXHI.	I303_14	:=		EXH_EL1889[4,14]	;
stEXHI.	I303_15	:=		EXH_EL1889[4,15]	;
stEXHI.	I304_00	:=		EXH_EL1889[5,0]	;
stEXHI. I304_01	:=		EXH_EL1889[5,1]	;
stEXHI. I304_02	:=		EXH_EL1889[5,2]	;
stEXHI. I304_03	:=		EXH_EL1889[5,3]	;
stEXHI. I304_04	:=		EXH_EL1889[5,4]	;
stEXHI. I304_05	:=		EXH_EL1889[5,5]	;
stEXHI. I304_06	:=		EXH_EL1889[5,6]	;
stEXHI. I304_07	:=		EXH_EL1889[5,7]	;
stEXHI. I304_08	:=		EXH_EL1889[5,8]	;
stEXHI. I304_09	:=		EXH_EL1889[5,9]	;
stEXHI. I304_10	:=		EXH_EL1889[5,10]	;
stEXHI. I304_11	:=		EXH_EL1889[5,11]	;
stEXHI. I304_12	:=		EXH_EL1889[5,12]	;
stEXHI. I304_13	:=		EXH_EL1889[5,13]	;
stEXHI. I304_14	:=		EXH_EL1889[5,14]	;
stEXHI. I304_15	:=		EXH_EL1889[5,15]	;

stEXHI.	IW300	:=		EXH_EL3124[1,	1]	;
stEXHI.	IW301	:=		EXH_EL3124[1,	2]	;
stEXHI.	IW302	:=		EXH_EL3124[1,	3]	;
stEXHI.	IW303	:=		EXH_EL3124[1,	4]	;
stEXHI.	IW304	:=		EXH_EL3124[2,	1]	;
stEXHI.	IW305	:=		EXH_EL3124[2,	2]	;
stEXHI.	IW306	:=		EXH_EL3124[2,	3]	;
stEXHI.	IW307	:=		EXH_EL3124[2,	4]	;
stEXHI.	IW308	:=		EXH_EL3124[3,	1]	;
stEXHI.	IW309	:=		EXH_EL3124[3,	2]	;
stEXHI.	IW310	:=		EXH_EL3124[3,	3]	;
stEXHI.	IW311	:=		EXH_EL3124[3,	4]	;
stEXHI.	IW312	:=		EXH_EL3124[4,	1]	;
stEXHI.	IW313	:=		EXH_EL3124[4,	2]	;
stEXHI.	IW314	:=		EXH_EL3124[4,	3]	;
stEXHI.	IW315	:=		EXH_EL3124[4,	4]	;
stEXHI.	IW316	:=		EXH_EL3164[1,	1]	;
stEXHI.	IW317	:=		EXH_EL3164[1,	2]	;
stEXHI.	IW318	:=		EXH_EL3164[1,	3]	;
stEXHI.	IW319	:=		EXH_EL3164[1,	4]	;
stEXHI.	IW320	:=		EXH_EL3164[2,	1]	;
stEXHI.	IW321	:=		EXH_EL3164[2,	2]	;
stEXHI.	IW322	:=		EXH_EL3164[2,	3]	;
stEXHI.	IW323	:=		EXH_EL3164[2,	4]	;
stEXHI.	IW324	:=		EXH_EL3164[3,	1]	;
stEXHI.	IW325	:=		EXH_EL3164[3,	2]	;
stEXHI.	IW326	:=		EXH_EL3164[3,	3]	;
stEXHI.	IW327	:=		EXH_EL3164[3,	4]	;
stEXHI.	IW328	:=		EXH_EL3164[4,	1]	;
stEXHI.	IW329	:=		EXH_EL3164[4,	2]	;
stEXHI.	IW330	:=		EXH_EL3164[4,	3]	;
stEXHI.	IW331	:=		EXH_EL3164[4,	4]	;
stEXHI.	IW332	:=		EXH_EL3124[5,	1]	;
stEXHI.	IW333	:=		EXH_EL3124[5,	2]	;
stEXHI.	IW334	:=		EXH_EL3124[5,	3]	;
stEXHI.	IW335	:=		EXH_EL3124[5,	4]	;

//************************************************************************
//06.OP Box INput/OUTPUT(天桥内PLC输入/出映射）
//************************************************************************
stOPI.	I600_00	:=		OP_EL1889[1,0]	;
stOPI.	I600_01	:=		OP_EL1889[1,1]	;
stOPI.	I600_02	:=		OP_EL1889[1,2]	;
stOPI.	I600_03	:=		OP_EL1889[1,3]	;
stOPI.	I600_04	:=		OP_EL1889[1,4]	;
stOPI.	I600_05	:=		OP_EL1889[1,5]	;
stOPI.	I600_06	:=		OP_EL1889[1,6]	;
stOPI.	I600_07	:=		OP_EL1889[1,7]	;
stOPI.	I600_08	:=		OP_EL1889[1,8]	;
stOPI.	I600_09	:=		OP_EL1889[1,9]	;
stOPI.	I600_10	:=		OP_EL1889[1,10]	;
stOPI.	I600_11	:=		OP_EL1889[1,11]	;
stOPI.	I600_12	:=		OP_EL1889[1,12]	;
stOPI.	I600_13	:=		OP_EL1889[1,13]	;
stOPI.	I600_14	:=		OP_EL1889[1,14]	;
stOPI.	I600_15	:=		OP_EL1889[1,15]	;

stOPI.	IW600	:=		OP_EL3124[1,	1]	;
stOPI.	IW601	:=		OP_EL3124[1,	2]	;
stOPI.	IW602	:=		OP_EL3124[1,	3]	;
stOPI.	IW603	:=		OP_EL3124[1,	4]	;
stOPI.	IW604	:=		OP_EL3124[2,	1]	;
stOPI.	IW605	:=		OP_EL3124[2,	2]	;
stOPI.	IW606	:=		OP_EL3124[2,	3]	;
stOPI.	IW607	:=		OP_EL3124[2,	4]	;
END_ACTION

ACTION Output:
//========================================================================
//!!!!!!!!!!!!!!!!!!!!以下依托于硬件，硬件无变动禁止更改!!!!!!!!!!!!!!!!!!
//=======================================================================

//************************************************************************
//02.Gas Box INput/OUTPUT(气体柜输入/出映射）
//************************************************************************
GB_EL2889[1,0]	:=	FALSE(*stGBQ.	Q200_00*)	;
GB_EL2889[1,1]	:=	stGBQ.	Q200_01	;
GB_EL2889[1,2]	:=	stGBQ.	Q200_02	;
GB_EL2889[1,3]	:=	stGBQ.	Q200_03	;
GB_EL2889[1,4]	:=	stGBQ.	Q200_04	;
GB_EL2889[1,5]	:=	stGBQ.	Q200_05	;
GB_EL2889[1,6]	:=	stGBQ.	Q200_06	;
GB_EL2889[1,7]	:=	stGBQ.	Q200_07	;
GB_EL2889[1,8]	:=	stGBQ.	Q200_08	;
GB_EL2889[1,9]	:=	stGBQ.	Q200_09	;
GB_EL2889[1,10]	:=	stGBQ.	Q200_10	;
GB_EL2889[1,11]	:=	stGBQ.	Q200_11	;
GB_EL2889[1,12]	:=	stGBQ.	Q200_12	;
GB_EL2889[1,13]	:=	stGBQ.	Q200_13	;
GB_EL2889[1,14]	:=	stGBQ.	Q200_14	;
GB_EL2889[1,15]	:=	stGBQ.	Q200_15	;

GB_EV := stGBQ.QEV ;

//************************************************************************
//03.EXH Box INput/OUTPUT(排气柜输入/出映射）
//************************************************************************
EXH_EL2889[1,0]		:=	NOT GVL.stPMCtoPLC.WAT_R_sw OR ( GVL.stPMCtoPLC.R_Axis_Temp > 80 ) (*stEXHQ.	Q300_00*)	;
EXH_EL2889[1,1]		:=	FALSE(*NOT GVL.stPMCtoPLC.WAT_F_sw OR 
						(	
							( GVL.stPMCtoPLC.Inlet_Ht_1_temp > 200) OR 
							( GVL.stPMCtoPLC.Inlet_Ht_2_temp > 200) OR
							( GVL.stPMCtoPLC.Port_Ht_1_temp > 200) 	OR
							( GVL.stPMCtoPLC.Port_Ht_2_temp > 200) 	OR
							( GVL.stPMCtoPLC.Port_Ht_3_temp > 200) 	OR
							( GVL.stPMCtoPLC.Port_Ht_4_temp > 200) 	OR
							( GVL.stPMCtoPLC.Port_Ht_5_temp > 200) 	
						)*)(*stEXHQ.	Q300_01*)	;
EXH_EL2889[1,2]		:=	stEXHQ.	Q300_02	;
EXH_EL2889[1,3]		:=	stEXHQ.	Q300_03	;
EXH_EL2889[1,4]		:=	stEXHQ.	Q300_04	;
EXH_EL2889[1,5]		:=	stEXHQ.	Q300_05	;
EXH_EL2889[1,6]		:=	stEXHQ.	Q300_06	;
EXH_EL2889[1,7]		:=	stEXHQ.	Q300_07	;
EXH_EL2889[1,8]		:=	TRUE(*stEXHQ.	Q300_08*) ;
EXH_EL2889[1,9]		:=	GVL.stPMCtoPLC.I103_00(*stEXHQ.	Q300_09*) ;
EXH_EL2889[1,10]	:=	TRUE(*stEXHQ.	Q300_10*) ;
EXH_EL2889[1,11]	:=	stEXHQ.	Q300_11	;
EXH_EL2889[1,12]	:=	stEXHQ.	Q300_12	;
EXH_EL2889[1,13]	:=	stEXHQ.	Q300_13	;
EXH_EL2889[1,14]	:=	stEXHQ.	Q300_14	;
EXH_EL2889[1,15]	:=	stEXHQ.	Q300_15	;

EXH_EV := stEXHQ.QEV ;
END_ACTION

ACTION PLC_to_PMC:
//Gas box
GVL.stPLCtoPMC.	I200_00	:=	stGBI.	I200_00	;
GVL.stPLCtoPMC.	I200_01	:=	stGBI.	I200_01	;
GVL.stPLCtoPMC.	I200_02	:=	stGBI.	I200_02	;
GVL.stPLCtoPMC.	I200_03	:=	stGBI.	I200_03	;
GVL.stPLCtoPMC.	I200_04	:=	stGBI.	I200_04	;
GVL.stPLCtoPMC.	I200_05	:=	stGBI.	I200_05	;
GVL.stPLCtoPMC.	I200_06	:=	stGBI.	I200_06	;
GVL.stPLCtoPMC.	I200_07	:=	stGBI.	I200_07	;
GVL.stPLCtoPMC.	I200_08	:=	stGBI.	I200_08	;
GVL.stPLCtoPMC.	I200_09	:=	stGBI.	I200_09	;
GVL.stPLCtoPMC.	I200_10	:=	stGBI.	I200_10	;
GVL.stPLCtoPMC.	I200_11	:=	stGBI.	I200_11	;
GVL.stPLCtoPMC.	I200_12	:=	stGBI.	I200_12	;
GVL.stPLCtoPMC.	I200_13	:=	stGBI.	I200_13	;
GVL.stPLCtoPMC.	I200_14	:=	stGBI.	I200_14	;
GVL.stPLCtoPMC.	I200_15	:=	stGBI.	I200_15	;
GVL.stPLCtoPMC.	I201_00	:=	stGBI.	I201_00	;
GVL.stPLCtoPMC.	I201_01	:=	stGBI.	I201_01	;
GVL.stPLCtoPMC.	I201_02	:=	stGBI.	I201_02	;
GVL.stPLCtoPMC.	I201_03	:=	stGBI.	I201_03	;
GVL.stPLCtoPMC.	I201_04	:=	stGBI.	I201_04	;
GVL.stPLCtoPMC.	I201_05	:=	stGBI.	I201_05	;
GVL.stPLCtoPMC.	I201_06	:=	stGBI.	I201_06	;
GVL.stPLCtoPMC.	I201_07	:=	stGBI.	I201_07	;
GVL.stPLCtoPMC.	I201_08	:=	stGBI.	I201_08	;
GVL.stPLCtoPMC.	I201_09	:=	stGBI.	I201_09	;
GVL.stPLCtoPMC.	I201_10	:=	stGBI.	I201_10	;
GVL.stPLCtoPMC.	I201_11	:=	stGBI.	I201_11	;
GVL.stPLCtoPMC.	I201_12	:=	stGBI.	I201_12	;
GVL.stPLCtoPMC.	I201_13	:=	stGBI.	I201_13	;
GVL.stPLCtoPMC.	I201_14	:=	stGBI.	I201_14	;
GVL.stPLCtoPMC.	I201_15	:=	stGBI.	I201_15	;
GVL.stPLCtoPMC.	I202_00	:=	stGBI.	I203_00	;
GVL.stPLCtoPMC.	I202_01	:=	stGBI.	I203_01	;
GVL.stPLCtoPMC.	I202_02	:=	stGBI.	I203_02	;
GVL.stPLCtoPMC.	I202_03	:=	stGBI.	I203_03	;
GVL.stPLCtoPMC.	I202_04	:=	stGBI.	I203_04	;
GVL.stPLCtoPMC.	I202_05	:=	stGBI.	I203_05	;
GVL.stPLCtoPMC.	I202_06	:=	stGBI.	I203_06	;
GVL.stPLCtoPMC.	I202_07	:=	stGBI.	I203_07	;
GVL.stPLCtoPMC.	I202_08	:=	stGBI.	I203_08	;
GVL.stPLCtoPMC.	I202_09	:=	stGBI.	I203_09	;
GVL.stPLCtoPMC.	I202_10	:=	stGBI.	I203_10	;
GVL.stPLCtoPMC.	I202_11	:=	stGBI.	I203_11	;
GVL.stPLCtoPMC.	I202_12	:=	stGBI.	I203_12	;
GVL.stPLCtoPMC.	I202_13	:=	stGBI.	I203_13	;
GVL.stPLCtoPMC.	I202_14	:=	stGBI.	I203_14	;
GVL.stPLCtoPMC.	I202_15	:=	stGBI.	I203_15	;

//Exhaust box
GVL.stPLCtoPMC.	I300_00	:=	stEXHI.	I300_00	;
GVL.stPLCtoPMC.	I300_01	:=	stEXHI.	I300_01	;
GVL.stPLCtoPMC.	I300_02	:=	stEXHI.	I300_02	;
GVL.stPLCtoPMC.	I300_03	:=	stEXHI.	I300_03	;
GVL.stPLCtoPMC.	I300_04	:=	stEXHI.	I300_04	;
GVL.stPLCtoPMC.	I300_05	:=	stEXHI.	I300_05	;
GVL.stPLCtoPMC.	I300_06	:=	stEXHI.	I300_06	;
GVL.stPLCtoPMC.	I300_07	:=	stEXHI.	I300_07	;
GVL.stPLCtoPMC.	I300_08	:=	stEXHI.	I300_08	;
GVL.stPLCtoPMC.	I300_09	:=	stEXHI.	I300_09	;
GVL.stPLCtoPMC.	I300_10	:=	stEXHI.	I300_10	;
GVL.stPLCtoPMC.	I300_11	:=	stEXHI.	I300_11	;
GVL.stPLCtoPMC.	I300_12	:=	stEXHI.	I300_12	;
GVL.stPLCtoPMC.	I300_13	:=	stEXHI.	I300_13	;
GVL.stPLCtoPMC.	I300_14	:=	stEXHI.	I300_14	;
GVL.stPLCtoPMC.	I300_15	:=	stEXHI.	I300_15	;
GVL.stPLCtoPMC.	I301_00	:=	stEXHI.	I301_00	;
GVL.stPLCtoPMC.	I301_01	:=	stEXHI.	I301_01	;
GVL.stPLCtoPMC.	I301_02	:=	stEXHI.	I301_02	;
GVL.stPLCtoPMC.	I301_03	:=	stEXHI.	I301_03	;
GVL.stPLCtoPMC.	I301_04	:=	stEXHI.	I301_04	;
GVL.stPLCtoPMC.	I301_05	:=	stEXHI.	I301_05	;
GVL.stPLCtoPMC.	I301_06	:=	stEXHI.	I301_06	;
GVL.stPLCtoPMC.	I301_07	:=	stEXHI.	I301_07	;
GVL.stPLCtoPMC.	I301_08	:=	stEXHI.	I301_08	;
GVL.stPLCtoPMC.	I301_09	:=	stEXHI.	I301_09	;
GVL.stPLCtoPMC.	I301_10	:=	stEXHI.	I301_10	;
GVL.stPLCtoPMC.	I301_11	:=	stEXHI.	I301_11	;
GVL.stPLCtoPMC.	I301_12	:=	stEXHI.	I301_12	;
GVL.stPLCtoPMC.	I301_13	:=	stEXHI.	I301_13	;
GVL.stPLCtoPMC.	I301_14	:=	stEXHI.	I301_14	;
GVL.stPLCtoPMC.	I301_15	:=	stEXHI.	I301_15	;
GVL.stPLCtoPMC.	I302_00	:=	stEXHI.	I302_00	;
GVL.stPLCtoPMC.	I302_01	:=	stEXHI.	I302_01	;
GVL.stPLCtoPMC.	I302_02	:=	stEXHI.	I302_02	;
GVL.stPLCtoPMC.	I302_03	:=	stEXHI.	I302_03	;
GVL.stPLCtoPMC.	I302_04	:=	stEXHI.	I302_04	;
GVL.stPLCtoPMC.	I302_05	:=	stEXHI.	I302_05	;
GVL.stPLCtoPMC.	I302_06	:=	stEXHI.	I302_06	;
GVL.stPLCtoPMC.	I302_07	:=	stEXHI.	I302_07	;
GVL.stPLCtoPMC.	I302_08	:=	stEXHI.	I302_08	;
GVL.stPLCtoPMC.	I302_09	:=	stEXHI.	I302_09	;
GVL.stPLCtoPMC.	I302_10	:=	stEXHI.	I302_10	;
GVL.stPLCtoPMC.	I302_11	:=	stEXHI.	I302_11	;
GVL.stPLCtoPMC.	I302_12	:=	stEXHI.	I302_12	;
GVL.stPLCtoPMC.	I302_13	:=	stEXHI.	I302_13	;
GVL.stPLCtoPMC.	I302_14	:=	stEXHI.	I302_14	;
GVL.stPLCtoPMC.	I302_15	:=	stEXHI.	I302_15	;
GVL.stPLCtoPMC.	I303_00	:=	stEXHI.	I303_00	;
GVL.stPLCtoPMC.	I303_01	:=	stEXHI.	I303_01	;
GVL.stPLCtoPMC.	I303_02	:=	stEXHI.	I303_02	;
GVL.stPLCtoPMC.	I303_03	:=	stEXHI.	I303_03	;
GVL.stPLCtoPMC.	I303_04	:=	stEXHI.	I303_04	;
GVL.stPLCtoPMC.	I303_05	:=	stEXHI.	I303_05	;
GVL.stPLCtoPMC.	I303_06	:=	stEXHI.	I303_06	;
GVL.stPLCtoPMC.	I303_07	:=	stEXHI.	I303_07	;
GVL.stPLCtoPMC.	I303_08	:=	stEXHI.	I303_08	;
GVL.stPLCtoPMC.	I303_09	:=	stEXHI.	I303_09	;
GVL.stPLCtoPMC.	I303_10	:=	stEXHI.	I303_10	;
GVL.stPLCtoPMC.	I303_11	:=	stEXHI.	I303_11	;
GVL.stPLCtoPMC.	I303_12	:=	stEXHI.	I303_12	;
GVL.stPLCtoPMC.	I303_13	:=	stEXHI.	I303_13	;
GVL.stPLCtoPMC.	I303_14	:=	stEXHI.	I303_14	;
GVL.stPLCtoPMC.	I303_15	:=	stEXHI.	I303_15	;
GVL.stPLCtoPMC.	I304_00	:=	stEXHI.	I304_00	;
GVL.stPLCtoPMC.	I304_01	:=	stEXHI.	I304_01	;
GVL.stPLCtoPMC.	I304_02	:=	stEXHI.	I304_02	;
GVL.stPLCtoPMC.	I304_03	:=	stEXHI.	I304_03	;
GVL.stPLCtoPMC.	I304_04	:=	stEXHI.	I304_04	;
GVL.stPLCtoPMC.	I304_05	:=	stEXHI.	I304_05	;
GVL.stPLCtoPMC.	I304_06	:=	stEXHI.	I304_06	;
GVL.stPLCtoPMC.	I304_07	:=	stEXHI.	I304_07	;
GVL.stPLCtoPMC.	I304_08	:=	stEXHI.	I304_08	;
GVL.stPLCtoPMC.	I304_09	:=	stEXHI.	I304_09	;
GVL.stPLCtoPMC.	I304_10	:=	stEXHI.	I304_10	;
GVL.stPLCtoPMC.	I304_11	:=	stEXHI.	I304_11	;
GVL.stPLCtoPMC.	I304_12	:=	stEXHI.	I304_12	;
GVL.stPLCtoPMC.	I304_13	:=	stEXHI.	I304_13	;
GVL.stPLCtoPMC.	I304_14	:=	stEXHI.	I304_14	;
GVL.stPLCtoPMC.	I304_15	:=	stEXHI.	I304_15	;

//Operation box
GVL.stPLCtoPMC.	I600_00	:=	stOPI.	I600_00	;
GVL.stPLCtoPMC.	I600_01	:=	stOPI.	I600_01	;
GVL.stPLCtoPMC.	I600_02	:=	stOPI.	I600_02	;
GVL.stPLCtoPMC.	I600_03	:=	stOPI.	I600_03	;
GVL.stPLCtoPMC.	I600_04	:=	stOPI.	I600_04	;
GVL.stPLCtoPMC.	I600_05	:=	stOPI.	I600_05	;
GVL.stPLCtoPMC.	I600_06	:=	stOPI.	I600_06	;
GVL.stPLCtoPMC.	I600_07	:=	stOPI.	I600_07	;
GVL.stPLCtoPMC.	I600_08	:=	stOPI.	I600_08	;
GVL.stPLCtoPMC.	I600_09	:=	stOPI.	I600_09	;
GVL.stPLCtoPMC.	I600_10	:=	stOPI.	I600_10	;
GVL.stPLCtoPMC.	I600_11	:=	stOPI.	I600_11	;
GVL.stPLCtoPMC.	I600_12	:=	stOPI.	I600_12	;
GVL.stPLCtoPMC.	I600_13	:=	stOPI.	I600_13	;
GVL.stPLCtoPMC.	I600_14	:=	stOPI.	I600_14	;
GVL.stPLCtoPMC.	I600_15	:=	stOPI.	I600_15	;

//FFU
GVL.stPLCtoPMC.	FFU1_1_STATUS	:=	UINT_TO_REAL(AI.	FFU1_1_STATUS	);
GVL.stPLCtoPMC.	FFU1_2_STATUS	:=	UINT_TO_REAL(AI.	FFU1_2_STATUS	);
GVL.stPLCtoPMC.	FFU1_3_STATUS	:=	UINT_TO_REAL(AI.	FFU1_3_STATUS	);
GVL.stPLCtoPMC.	FFU1_4_STATUS	:=	UINT_TO_REAL(AI.	FFU1_4_STATUS	);
GVL.stPLCtoPMC.	FFU1_5_STATUS	:=	UINT_TO_REAL(AI.	FFU1_5_STATUS	);
GVL.stPLCtoPMC.	FFU1_6_STATUS	:=	UINT_TO_REAL(AI.	FFU1_6_STATUS	);
GVL.stPLCtoPMC.	FFU2_1_STATUS	:=	UINT_TO_REAL(AI.	FFU2_1_STATUS	);
GVL.stPLCtoPMC.	FFU2_2_STATUS	:=	UINT_TO_REAL(AI.	FFU2_2_STATUS	);
GVL.stPLCtoPMC.	FFU2_3_STATUS	:=	UINT_TO_REAL(AI.	FFU2_3_STATUS	);
GVL.stPLCtoPMC.	FFU2_4_STATUS	:=	UINT_TO_REAL(AI.	FFU2_4_STATUS	);
GVL.stPLCtoPMC.	FFU2_5_STATUS	:=	UINT_TO_REAL(AI.	FFU2_5_STATUS	);
GVL.stPLCtoPMC.	FFU2_6_STATUS	:=	UINT_TO_REAL(AI.	FFU2_6_STATUS	);
GVL.stPLCtoPMC.	FFU3_1_STATUS	:=	UINT_TO_REAL(AI.	FFU3_1_STATUS	);
GVL.stPLCtoPMC.	FFU3_2_STATUS	:=	UINT_TO_REAL(AI.	FFU3_2_STATUS	);
GVL.stPLCtoPMC.	FFU3_3_STATUS	:=	UINT_TO_REAL(AI.	FFU3_3_STATUS	);
GVL.stPLCtoPMC.	FFU3_4_STATUS	:=	UINT_TO_REAL(AI.	FFU3_4_STATUS	);
GVL.stPLCtoPMC.	FFU3_5_STATUS	:=	UINT_TO_REAL(AI.	FFU3_5_STATUS	);
GVL.stPLCtoPMC.	FFU3_6_STATUS	:=	UINT_TO_REAL(AI.	FFU3_6_STATUS	);

GVL.stPLCtoPMC.	FFU1_1_SPEED_PV	:=	UINT_TO_REAL(AI.	FFU1_1_SPEED_PV	);
GVL.stPLCtoPMC.	FFU1_2_SPEED_PV	:=	UINT_TO_REAL(AI.	FFU1_2_SPEED_PV	);
GVL.stPLCtoPMC.	FFU1_3_SPEED_PV	:=	UINT_TO_REAL(AI.	FFU1_3_SPEED_PV	);
GVL.stPLCtoPMC.	FFU1_4_SPEED_PV	:=	UINT_TO_REAL(AI.	FFU1_4_SPEED_PV	);
GVL.stPLCtoPMC.	FFU1_5_SPEED_PV	:=	UINT_TO_REAL(AI.	FFU1_5_SPEED_PV	);
GVL.stPLCtoPMC.	FFU1_6_SPEED_PV	:=	UINT_TO_REAL(AI.	FFU1_6_SPEED_PV	);
GVL.stPLCtoPMC.	FFU2_1_SPEED_PV	:=	UINT_TO_REAL(AI.	FFU2_1_SPEED_PV	);
GVL.stPLCtoPMC.	FFU2_2_SPEED_PV	:=	UINT_TO_REAL(AI.	FFU2_2_SPEED_PV	);
GVL.stPLCtoPMC.	FFU2_3_SPEED_PV	:=	UINT_TO_REAL(AI.	FFU2_3_SPEED_PV	);
GVL.stPLCtoPMC.	FFU2_4_SPEED_PV	:=	UINT_TO_REAL(AI.	FFU2_4_SPEED_PV	);
GVL.stPLCtoPMC.	FFU2_5_SPEED_PV	:=	UINT_TO_REAL(AI.	FFU2_5_SPEED_PV	);
GVL.stPLCtoPMC.	FFU2_6_SPEED_PV	:=	UINT_TO_REAL(AI.	FFU2_6_SPEED_PV	);
GVL.stPLCtoPMC.	FFU3_1_SPEED_PV	:=	UINT_TO_REAL(AI.	FFU3_1_SPEED_PV	);
GVL.stPLCtoPMC.	FFU3_2_SPEED_PV	:=	UINT_TO_REAL(AI.	FFU3_2_SPEED_PV	);
GVL.stPLCtoPMC.	FFU3_3_SPEED_PV	:=	UINT_TO_REAL(AI.	FFU3_3_SPEED_PV	);
GVL.stPLCtoPMC.	FFU3_4_SPEED_PV	:=	UINT_TO_REAL(AI.	FFU3_4_SPEED_PV	);
GVL.stPLCtoPMC.	FFU3_5_SPEED_PV	:=	UINT_TO_REAL(AI.	FFU3_5_SPEED_PV	);
GVL.stPLCtoPMC.	FFU3_6_SPEED_PV	:=	UINT_TO_REAL(AI.	FFU3_6_SPEED_PV	);
END_ACTION

ACTION PMC_to_PLC:
//Gas box
stGBQ.	Q200_00	:=	GVL.stPMCtoPLC.	Q200_00	;
stGBQ.	Q200_01	:=	GVL.stPMCtoPLC.	Q200_01	;
stGBQ.	Q200_02	:=	GVL.stPMCtoPLC.	Q200_02	;
stGBQ.	Q200_03	:=	GVL.stPMCtoPLC.	Q200_03	;
stGBQ.	Q200_04	:=	GVL.stPMCtoPLC.	Q200_04	;
stGBQ.	Q200_05	:=	GVL.stPMCtoPLC.	Q200_05	;
stGBQ.	Q200_06	:=	GVL.stPMCtoPLC.	Q200_06	;
stGBQ.	Q200_07	:=	GVL.stPMCtoPLC.	Q200_07	;
stGBQ.	Q200_08	:=	GVL.stPMCtoPLC.	Q200_08	;
stGBQ.	Q200_09	:=	GVL.stPMCtoPLC.	Q200_09	;
stGBQ.	Q200_10	:=	GVL.stPMCtoPLC.	Q200_10	;
stGBQ.	Q200_11	:=	GVL.stPMCtoPLC.	Q200_11	;
stGBQ.	Q200_12	:=	GVL.stPMCtoPLC.	Q200_12	;
stGBQ.	Q200_13	:=	GVL.stPMCtoPLC.	Q200_13	;
stGBQ.	Q200_14	:=	GVL.stPMCtoPLC.	Q200_14	;
stGBQ.	Q200_15	:=	GVL.stPMCtoPLC.	Q200_15	;

//Exhaust box
stEXHQ.	Q300_00	:=	GVL.stPMCtoPLC.	Q300_00	;
stEXHQ.	Q300_01	:=	GVL.stPMCtoPLC.	Q300_01	;
stEXHQ.	Q300_02	:=	GVL.stPMCtoPLC.	Q300_02	;
stEXHQ.	Q300_03	:=	GVL.stPMCtoPLC.	Q300_03	;
stEXHQ.	Q300_04	:=	GVL.stPMCtoPLC.	Q300_04	;
stEXHQ.	Q300_05	:=	GVL.stPMCtoPLC.	Q300_05	;
stEXHQ.	Q300_06	:=	GVL.stPMCtoPLC.	Q300_06	;
stEXHQ.	Q300_07	:=	GVL.stPMCtoPLC.	Q300_07	;
stEXHQ.	Q300_08	:=	GVL.stPMCtoPLC.	Q300_08	;
stEXHQ.	Q300_09	:=	GVL.stPMCtoPLC.	Q300_09	;
stEXHQ.	Q300_10	:=	GVL.stPMCtoPLC.	Q300_10	;
stEXHQ.	Q300_11	:=	GVL.stPMCtoPLC.	Q300_11	;
stEXHQ.	Q300_12	:=	GVL.stPMCtoPLC.	Q300_12	;
stEXHQ.	Q300_13	:=	GVL.stPMCtoPLC.	Q300_13	;
stEXHQ.	Q300_14	:=	GVL.stPMCtoPLC.	Q300_14	;
stEXHQ.	Q300_15	:=	GVL.stPMCtoPLC.	Q300_15	;

//FFU
AO.	FFU_ALARM_EN	:=	REAL_TO_UINT(GVL.stPMCtoPLC.	FFU_ALARM_EN	);
AO.	FFU_HSPEED		:=	REAL_TO_UINT(GVL.stPMCtoPLC.	FFU_HSPEED		);
AO.	FFU_LSPEED		:=	REAL_TO_UINT(GVL.stPMCtoPLC.	FFU_LSPEED		);
AO.	FFU1_1_POWER_ON	:=	REAL_TO_UINT(GVL.stPMCtoPLC.	FFU1_1_POWER_ON	);
AO.	FFU1_2_POWER_ON	:=	REAL_TO_UINT(GVL.stPMCtoPLC.	FFU1_2_POWER_ON	);
AO.	FFU1_3_POWER_ON	:=	REAL_TO_UINT(GVL.stPMCtoPLC.	FFU1_3_POWER_ON	);
AO.	FFU1_4_POWER_ON	:=	REAL_TO_UINT(GVL.stPMCtoPLC.	FFU1_4_POWER_ON	);
AO.	FFU1_5_POWER_ON	:=	REAL_TO_UINT(GVL.stPMCtoPLC.	FFU1_5_POWER_ON	);
AO.	FFU1_6_POWER_ON	:=	REAL_TO_UINT(GVL.stPMCtoPLC.	FFU1_6_POWER_ON	);
AO.	FFU2_1_POWER_ON	:=	REAL_TO_UINT(GVL.stPMCtoPLC.	FFU2_1_POWER_ON	);
AO.	FFU2_2_POWER_ON	:=	REAL_TO_UINT(GVL.stPMCtoPLC.	FFU2_2_POWER_ON	);
AO.	FFU2_3_POWER_ON	:=	REAL_TO_UINT(GVL.stPMCtoPLC.	FFU2_3_POWER_ON	);
AO.	FFU2_4_POWER_ON	:=	REAL_TO_UINT(GVL.stPMCtoPLC.	FFU2_4_POWER_ON	);
AO.	FFU2_5_POWER_ON	:=	REAL_TO_UINT(GVL.stPMCtoPLC.	FFU2_5_POWER_ON	);
AO.	FFU2_6_POWER_ON	:=	REAL_TO_UINT(GVL.stPMCtoPLC.	FFU2_6_POWER_ON	);
AO.	FFU3_1_POWER_ON	:=	REAL_TO_UINT(GVL.stPMCtoPLC.	FFU3_1_POWER_ON	);
AO.	FFU3_2_POWER_ON	:=	REAL_TO_UINT(GVL.stPMCtoPLC.	FFU3_2_POWER_ON	);
AO.	FFU3_3_POWER_ON	:=	REAL_TO_UINT(GVL.stPMCtoPLC.	FFU3_3_POWER_ON	);
AO.	FFU3_4_POWER_ON	:=	REAL_TO_UINT(GVL.stPMCtoPLC.	FFU3_4_POWER_ON	);
AO.	FFU3_5_POWER_ON	:=	REAL_TO_UINT(GVL.stPMCtoPLC.	FFU3_5_POWER_ON	);
AO.	FFU3_6_POWER_ON	:=	REAL_TO_UINT(GVL.stPMCtoPLC.	FFU3_6_POWER_ON	);
AO.	FFU1_1_SPEED_SV	:=	REAL_TO_UINT(GVL.stPMCtoPLC.	FFU1_1_SPEED_SV	);
AO.	FFU1_2_SPEED_SV	:=	REAL_TO_UINT(GVL.stPMCtoPLC.	FFU1_2_SPEED_SV	);
AO.	FFU1_3_SPEED_SV	:=	REAL_TO_UINT(GVL.stPMCtoPLC.	FFU1_3_SPEED_SV	);
AO.	FFU1_4_SPEED_SV	:=	REAL_TO_UINT(GVL.stPMCtoPLC.	FFU1_4_SPEED_SV	);
AO.	FFU1_5_SPEED_SV	:=	REAL_TO_UINT(GVL.stPMCtoPLC.	FFU1_5_SPEED_SV	);
AO.	FFU1_6_SPEED_SV	:=	REAL_TO_UINT(GVL.stPMCtoPLC.	FFU1_6_SPEED_SV	);
AO.	FFU2_1_SPEED_SV	:=	REAL_TO_UINT(GVL.stPMCtoPLC.	FFU2_1_SPEED_SV	);
AO.	FFU2_2_SPEED_SV	:=	REAL_TO_UINT(GVL.stPMCtoPLC.	FFU2_2_SPEED_SV	);
AO.	FFU2_3_SPEED_SV	:=	REAL_TO_UINT(GVL.stPMCtoPLC.	FFU2_3_SPEED_SV	);
AO.	FFU2_4_SPEED_SV	:=	REAL_TO_UINT(GVL.stPMCtoPLC.	FFU2_4_SPEED_SV	);
AO.	FFU2_5_SPEED_SV	:=	REAL_TO_UINT(GVL.stPMCtoPLC.	FFU2_5_SPEED_SV	);
AO.	FFU2_6_SPEED_SV	:=	REAL_TO_UINT(GVL.stPMCtoPLC.	FFU2_6_SPEED_SV	);
AO.	FFU3_1_SPEED_SV	:=	REAL_TO_UINT(GVL.stPMCtoPLC.	FFU3_1_SPEED_SV	);
AO.	FFU3_2_SPEED_SV	:=	REAL_TO_UINT(GVL.stPMCtoPLC.	FFU3_2_SPEED_SV	);
AO.	FFU3_3_SPEED_SV	:=	REAL_TO_UINT(GVL.stPMCtoPLC.	FFU3_3_SPEED_SV	);
AO.	FFU3_4_SPEED_SV	:=	REAL_TO_UINT(GVL.stPMCtoPLC.	FFU3_4_SPEED_SV	);
AO.	FFU3_5_SPEED_SV	:=	REAL_TO_UINT(GVL.stPMCtoPLC.	FFU3_5_SPEED_SV	);
AO.	FFU3_6_SPEED_SV	:=	REAL_TO_UINT(GVL.stPMCtoPLC.	FFU3_6_SPEED_SV	);
AO.	FFU1_1_EN		:=	REAL_TO_UINT(GVL.stPMCtoPLC.	FFU1_1_EN		);
AO.	FFU1_2_EN		:=	REAL_TO_UINT(GVL.stPMCtoPLC.	FFU1_2_EN		);
AO.	FFU1_3_EN		:=	REAL_TO_UINT(GVL.stPMCtoPLC.	FFU1_3_EN		);
AO.	FFU1_4_EN		:=	REAL_TO_UINT(GVL.stPMCtoPLC.	FFU1_4_EN		);
AO.	FFU1_5_EN		:=	REAL_TO_UINT(GVL.stPMCtoPLC.	FFU1_5_EN		);
AO.	FFU1_6_EN		:=	REAL_TO_UINT(GVL.stPMCtoPLC.	FFU1_6_EN		);
AO.	FFU2_1_EN		:=	REAL_TO_UINT(GVL.stPMCtoPLC.	FFU2_1_EN		);
AO.	FFU2_2_EN		:=	REAL_TO_UINT(GVL.stPMCtoPLC.	FFU2_2_EN		);
AO.	FFU2_3_EN		:=	REAL_TO_UINT(GVL.stPMCtoPLC.	FFU2_3_EN		);
AO.	FFU2_4_EN		:=	REAL_TO_UINT(GVL.stPMCtoPLC.	FFU2_4_EN		);
AO.	FFU2_5_EN		:=	REAL_TO_UINT(GVL.stPMCtoPLC.	FFU2_5_EN		);
AO.	FFU2_6_EN		:=	REAL_TO_UINT(GVL.stPMCtoPLC.	FFU2_6_EN		);
AO.	FFU3_1_EN		:=	REAL_TO_UINT(GVL.stPMCtoPLC.	FFU3_1_EN		);
AO.	FFU3_2_EN		:=	REAL_TO_UINT(GVL.stPMCtoPLC.	FFU3_2_EN		);
AO.	FFU3_3_EN		:=	REAL_TO_UINT(GVL.stPMCtoPLC.	FFU3_3_EN		);
AO.	FFU3_4_EN		:=	REAL_TO_UINT(GVL.stPMCtoPLC.	FFU3_4_EN		);
AO.	FFU3_5_EN		:=	REAL_TO_UINT(GVL.stPMCtoPLC.	FFU3_5_EN		);
AO.	FFU3_6_EN		:=	REAL_TO_UINT(GVL.stPMCtoPLC.	FFU3_6_EN		);
END_ACTION

ACTION ValveCtrl:
//EMO status
bEMOStatus := 
	GVL.stPMCtoPLC.EMO101_power_box_EMO AND GVL.stPMCtoPLC.EMO301_Exhaust_box_EMO AND GVL.stPMCtoPLC.EMO401_frontbody_EMO AND
	GVL.stPMCtoPLC.SMK1_detector_operator AND GVL.stPMCtoPLC.Power_box_fire_detector_alarm ;

AV[1]				
(	bValveEnable_In 	:= TRUE ,		
	bInterlock1_In		:= bEMOStatus ,	
	bInterlock2_In		:= TRUE ,	
	bInterlock3_In		:= TRUE ,	
	bInterlock4_In		:= TRUE ,	
	bInterlock5_In		:= TRUE ,	
	bForceOpen_In		:= aForceOpValve[1],
	bValveInterlock_In	:= aILK_AV[1] ,		
	bPMCCtrl_In			:= GVL.stPMCtoPLC.aAV[1] ,
	bValveOpen_Out		=> aAV[1] 
);				
				
AV[2]				
(	bValveEnable_In 	:= TRUE ,		
	bInterlock1_In		:= bEMOStatus ,	
	bInterlock2_In		:= TRUE ,	
	bInterlock3_In		:= TRUE ,	
	bInterlock4_In		:= TRUE ,	
	bInterlock5_In		:= TRUE ,	
	bForceOpen_In		:= aForceOpValve[2],
	bValveInterlock_In	:= aILK_AV[2] ,		
	bPMCCtrl_In			:= GVL.stPMCtoPLC.aAV[2] ,
	bValveOpen_Out		=> aAV[2] 	
);				
				
AV[3]				
(	bValveEnable_In 	:= TRUE ,		
	bInterlock1_In		:= bEMOStatus ,	
	bInterlock2_In		:= TRUE ,	
	bInterlock3_In		:= TRUE ,	
	bInterlock4_In		:= TRUE ,	
	bInterlock5_In		:= TRUE ,	
	bForceOpen_In		:= aForceOpValve[3],
	bValveInterlock_In	:= aILK_AV[3] ,		
	bPMCCtrl_In			:= GVL.stPMCtoPLC.aAV[3] ,
	bValveOpen_Out		=> aAV[3] 	
);				
				
AV[4]				
(	bValveEnable_In 	:= TRUE ,		
	bInterlock1_In		:= bEMOStatus ,	
	bInterlock2_In		:= TRUE ,	
	bInterlock3_In		:= TRUE ,	
	bInterlock4_In		:= TRUE ,	
	bInterlock5_In		:= TRUE ,	
	bForceOpen_In		:= aForceOpValve[4],
	bValveInterlock_In	:= aILK_AV[4] ,		
	bPMCCtrl_In			:= GVL.stPMCtoPLC.aAV[4] ,
	bValveOpen_Out		=> aAV[4] 	
);				
				
AV[5]				
(	bValveEnable_In 	:= TRUE ,		
	bInterlock1_In		:= bEMOStatus ,	
	bInterlock2_In		:= TRUE ,	
	bInterlock3_In		:= TRUE ,	
	bInterlock4_In		:= TRUE ,	
	bInterlock5_In		:= TRUE ,	
	bForceOpen_In		:= aForceOpValve[5],
	bValveInterlock_In	:= aILK_AV[5] ,		
	bPMCCtrl_In			:= GVL.stPMCtoPLC.aAV[5] ,
	bValveOpen_Out		=> aAV[5] 	
);				
				
AV[6]				
(	bValveEnable_In 	:= TRUE ,		
	bInterlock1_In		:= bEMOStatus ,	
	bInterlock2_In		:= TRUE ,	
	bInterlock3_In		:= TRUE ,	
	bInterlock4_In		:= TRUE ,	
	bInterlock5_In		:= TRUE ,	
	bForceOpen_In		:= aForceOpValve[6],
	bValveInterlock_In	:= aILK_AV[6] ,		
	bPMCCtrl_In			:= GVL.stPMCtoPLC.aAV[6] ,
	bValveOpen_Out		=> aAV[6] 	
);				
				
AV[7]				
(	bValveEnable_In 	:= TRUE ,		
	bInterlock1_In		:= bEMOStatus ,	
	bInterlock2_In		:= TRUE ,	
	bInterlock3_In		:= TRUE ,	
	bInterlock4_In		:= TRUE ,	
	bInterlock5_In		:= TRUE ,	
	bForceOpen_In		:= aForceOpValve[7],
	bValveInterlock_In	:= aILK_AV[7] ,		
	bPMCCtrl_In			:= GVL.stPMCtoPLC.aAV[7] ,
	bValveOpen_Out		=> aAV[7] 	
);				
				
AV[8]				
(	bValveEnable_In 	:= TRUE ,		
	bInterlock1_In		:= bEMOStatus ,	
	bInterlock2_In		:= TRUE ,	
	bInterlock3_In		:= TRUE ,	
	bInterlock4_In		:= TRUE ,	
	bInterlock5_In		:= TRUE ,	
	bForceOpen_In		:= aForceOpValve[8],
	bValveInterlock_In	:= aILK_AV[8] ,		
	bPMCCtrl_In			:= GVL.stPMCtoPLC.aAV[8] ,
	bValveOpen_Out		=> aAV[8] 	
);				
				
AV[9]				
(	bValveEnable_In 	:= TRUE ,		
	bInterlock1_In		:= bEMOStatus ,	
	bInterlock2_In		:= TRUE ,	
	bInterlock3_In		:= TRUE ,	
	bInterlock4_In		:= TRUE ,	
	bInterlock5_In		:= TRUE ,	
	bForceOpen_In		:= aForceOpValve[9],
	bValveInterlock_In	:= aILK_AV[9] ,		
	bPMCCtrl_In			:= GVL.stPMCtoPLC.aAV[9] ,
	bValveOpen_Out		=> aAV[9] 	
);				
				
AV[10]				
(	bValveEnable_In 	:= TRUE ,		
	bInterlock1_In		:= bEMOStatus ,	
	bInterlock2_In		:= TRUE ,	
	bInterlock3_In		:= TRUE ,	
	bInterlock4_In		:= TRUE ,	
	bInterlock5_In		:= TRUE ,	
	bForceOpen_In		:= aForceOpValve[10],
	bValveInterlock_In	:= aILK_AV[10] ,		
	bPMCCtrl_In			:= GVL.stPMCtoPLC.aAV[10] ,
	bValveOpen_Out		=> aAV[10] 	
);				
				
AV[11]				
(	bValveEnable_In 	:= TRUE ,		
	bInterlock1_In		:= bEMOStatus ,	
	bInterlock2_In		:= TRUE ,	
	bInterlock3_In		:= TRUE ,	
	bInterlock4_In		:= TRUE ,	
	bInterlock5_In		:= TRUE ,	
	bForceOpen_In		:= aForceOpValve[11],
	bValveInterlock_In	:= aILK_AV[11] ,		
	bPMCCtrl_In			:= GVL.stPMCtoPLC.aAV[11] ,
	bValveOpen_Out		=> aAV[11] 	
);				
				
AV[12]				
(	bValveEnable_In 	:= TRUE ,		
	bInterlock1_In		:= bEMOStatus ,	
	bInterlock2_In		:= TRUE ,	
	bInterlock3_In		:= TRUE ,	
	bInterlock4_In		:= TRUE ,	
	bInterlock5_In		:= TRUE ,	
	bForceOpen_In		:= aForceOpValve[12],
	bValveInterlock_In	:= aILK_AV[12] ,		
	bPMCCtrl_In			:= GVL.stPMCtoPLC.aAV[12] ,
	bValveOpen_Out		=> aAV[12] 	
);				
				
AV[13]				
(	bValveEnable_In 	:= TRUE ,		
	bInterlock1_In		:= bEMOStatus ,	
	bInterlock2_In		:= TRUE ,	
	bInterlock3_In		:= TRUE ,	
	bInterlock4_In		:= TRUE ,	
	bInterlock5_In		:= TRUE ,	
	bForceOpen_In		:= aForceOpValve[13],
	bValveInterlock_In	:= aILK_AV[13] ,		
	bPMCCtrl_In			:= GVL.stPMCtoPLC.aAV[13] ,
	bValveOpen_Out		=> aAV[13] 	
);				
				
AV[14]				
(	bValveEnable_In 	:= TRUE ,		
	bInterlock1_In		:= bEMOStatus ,	
	bInterlock2_In		:= TRUE ,	
	bInterlock3_In		:= TRUE ,	
	bInterlock4_In		:= TRUE ,	
	bInterlock5_In		:= TRUE ,	
	bForceOpen_In		:= aForceOpValve[14],
	bValveInterlock_In	:= aILK_AV[14] ,		
	bPMCCtrl_In			:= GVL.stPMCtoPLC.aAV[14] ,
	bValveOpen_Out		=> aAV[14] 	
);				
				
AV[15]				
(	bValveEnable_In 	:= TRUE ,		
	bInterlock1_In		:= bEMOStatus ,	
	bInterlock2_In		:= TRUE ,	
	bInterlock3_In		:= TRUE ,	
	bInterlock4_In		:= TRUE ,	
	bInterlock5_In		:= TRUE ,	
	bForceOpen_In		:= aForceOpValve[15],
	bValveInterlock_In	:= aILK_AV[15] ,		
	bPMCCtrl_In			:= GVL.stPMCtoPLC.aAV[15] ,
	bValveOpen_Out		=> aAV[15] 	
);				
				
AV[16]				
(	bValveEnable_In 	:= TRUE ,		
	bInterlock1_In		:= bEMOStatus ,	
	bInterlock2_In		:= TRUE ,	
	bInterlock3_In		:= TRUE ,	
	bInterlock4_In		:= TRUE ,	
	bInterlock5_In		:= TRUE ,	
	bForceOpen_In		:= aForceOpValve[16],
	bValveInterlock_In	:= aILK_AV[16] ,		
	bPMCCtrl_In			:= GVL.stPMCtoPLC.aAV[16] ,
	bValveOpen_Out		=> aAV[16] 	
);				
				
AV[17]				
(	bValveEnable_In 	:= TRUE ,		
	bInterlock1_In		:= bEMOStatus ,	
	bInterlock2_In		:= TRUE ,	
	bInterlock3_In		:= TRUE ,	
	bInterlock4_In		:= TRUE ,	
	bInterlock5_In		:= TRUE ,	
	bForceOpen_In		:= aForceOpValve[17],
	bValveInterlock_In	:= aILK_AV[17] ,		
	bPMCCtrl_In			:= GVL.stPMCtoPLC.aAV[17] ,
	bValveOpen_Out		=> aAV[17] 	
);				
				
AV[18]				
(	bValveEnable_In 	:= TRUE ,		
	bInterlock1_In		:= bEMOStatus ,	
	bInterlock2_In		:= TRUE ,	
	bInterlock3_In		:= TRUE ,	
	bInterlock4_In		:= TRUE ,	
	bInterlock5_In		:= TRUE ,	
	bForceOpen_In		:= aForceOpValve[18],
	bValveInterlock_In	:= aILK_AV[18] ,		
	bPMCCtrl_In			:= GVL.stPMCtoPLC.aAV[18] ,
	bValveOpen_Out		=> aAV[18] 	
);				
				
AV[19]				
(	bValveEnable_In 	:= TRUE ,		
	bInterlock1_In		:= bEMOStatus ,	
	bInterlock2_In		:= TRUE ,	
	bInterlock3_In		:= TRUE ,	
	bInterlock4_In		:= TRUE ,	
	bInterlock5_In		:= TRUE ,	
	bForceOpen_In		:= aForceOpValve[19],
	bValveInterlock_In	:= aILK_AV[19] ,		
	bPMCCtrl_In			:= GVL.stPMCtoPLC.aAV[19] ,
	bValveOpen_Out		=> aAV[19] 	
);				
				
AV[20]				
(	bValveEnable_In 	:= TRUE ,		
	bInterlock1_In		:= bEMOStatus ,	
	bInterlock2_In		:= TRUE ,	
	bInterlock3_In		:= TRUE ,	
	bInterlock4_In		:= TRUE ,	
	bInterlock5_In		:= TRUE ,	
	bForceOpen_In		:= aForceOpValve[20],
	bValveInterlock_In	:= aILK_AV[20] ,		
	bPMCCtrl_In			:= GVL.stPMCtoPLC.aAV[20] ,
	bValveOpen_Out		=> aAV[20] 	
);				
				
AV[21]				
(	bValveEnable_In 	:= TRUE ,		
	bInterlock1_In		:= bEMOStatus ,	
	bInterlock2_In		:= TRUE ,	
	bInterlock3_In		:= TRUE ,	
	bInterlock4_In		:= TRUE ,	
	bInterlock5_In		:= TRUE ,	
	bForceOpen_In		:= aForceOpValve[21],
	bValveInterlock_In	:= aILK_AV[21] ,		
	bPMCCtrl_In			:= GVL.stPMCtoPLC.aAV[21] ,
	bValveOpen_Out		=> aAV[21] 	
);				
				
AV[22]				
(	bValveEnable_In 	:= TRUE ,		
	bInterlock1_In		:= bEMOStatus ,	
	bInterlock2_In		:= TRUE ,	
	bInterlock3_In		:= TRUE ,	
	bInterlock4_In		:= TRUE ,	
	bInterlock5_In		:= TRUE ,	
	bForceOpen_In		:= aForceOpValve[22],
	bValveInterlock_In	:= aILK_AV[22] ,		
	bPMCCtrl_In			:= GVL.stPMCtoPLC.aAV[22] ,
	bValveOpen_Out		=> aAV[22] 	
);				
				
AV[23]				
(	bValveEnable_In 	:= TRUE ,		
	bInterlock1_In		:= bEMOStatus ,	
	bInterlock2_In		:= TRUE ,	
	bInterlock3_In		:= TRUE ,	
	bInterlock4_In		:= TRUE ,	
	bInterlock5_In		:= TRUE ,	
	bForceOpen_In		:= aForceOpValve[23],
	bValveInterlock_In	:= aILK_AV[23] ,		
	bPMCCtrl_In			:= GVL.stPMCtoPLC.aAV[23] ,
	bValveOpen_Out		=> aAV[23] 	
);				
				
AV[24]				
(	bValveEnable_In 	:= TRUE ,		
	bInterlock1_In		:= bEMOStatus ,	
	bInterlock2_In		:= TRUE ,	
	bInterlock3_In		:= TRUE ,	
	bInterlock4_In		:= TRUE ,	
	bInterlock5_In		:= TRUE ,	
	bForceOpen_In		:= aForceOpValve[24],
	bValveInterlock_In	:= aILK_AV[24] ,		
	bPMCCtrl_In			:= GVL.stPMCtoPLC.aAV[24] ,
	bValveOpen_Out		=> aAV[24] 	
);				
				
AV[25]				
(	bValveEnable_In 	:= TRUE ,		
	bInterlock1_In		:= bEMOStatus ,	
	bInterlock2_In		:= TRUE ,	
	bInterlock3_In		:= TRUE ,	
	bInterlock4_In		:= TRUE ,	
	bInterlock5_In		:= TRUE ,	
	bForceOpen_In		:= aForceOpValve[25],
	bValveInterlock_In	:= aILK_AV[25] ,		
	bPMCCtrl_In			:= GVL.stPMCtoPLC.aAV[25] ,
	bValveOpen_Out		=> aAV[25] 	
);				
				
AV[26]				
(	bValveEnable_In 	:= TRUE ,		
	bInterlock1_In		:= bEMOStatus ,	
	bInterlock2_In		:= TRUE ,	
	bInterlock3_In		:= TRUE ,	
	bInterlock4_In		:= TRUE ,	
	bInterlock5_In		:= TRUE ,	
	bForceOpen_In		:= aForceOpValve[26],
	bValveInterlock_In	:= aILK_AV[26] ,		
	bPMCCtrl_In			:= GVL.stPMCtoPLC.aAV[26] ,
	bValveOpen_Out		=> aAV[26] 	
);				
				
AV[27]				
(	bValveEnable_In 	:= TRUE ,		
	bInterlock1_In		:= bEMOStatus ,	
	bInterlock2_In		:= TRUE ,	
	bInterlock3_In		:= TRUE ,	
	bInterlock4_In		:= TRUE ,	
	bInterlock5_In		:= TRUE ,	
	bForceOpen_In		:= aForceOpValve[27],
	bValveInterlock_In	:= aILK_AV[27] ,		
	bPMCCtrl_In			:= GVL.stPMCtoPLC.aAV[27] ,
	bValveOpen_Out		=> aAV[27] 	
);				
				
AV[28]				
(	bValveEnable_In 	:= TRUE ,		
	bInterlock1_In		:= bEMOStatus ,	
	bInterlock2_In		:= TRUE ,	
	bInterlock3_In		:= TRUE ,	
	bInterlock4_In		:= TRUE ,	
	bInterlock5_In		:= TRUE ,	
	bForceOpen_In		:= aForceOpValve[28],
	bValveInterlock_In	:= aILK_AV[28] ,		
	bPMCCtrl_In			:= GVL.stPMCtoPLC.aAV[28] ,
	bValveOpen_Out		=> aAV[28] 	
);				
				
AV[29]				
(	bValveEnable_In 	:= TRUE ,		
	bInterlock1_In		:= bEMOStatus ,	
	bInterlock2_In		:= TRUE ,	
	bInterlock3_In		:= TRUE ,	
	bInterlock4_In		:= TRUE ,	
	bInterlock5_In		:= TRUE ,	
	bForceOpen_In		:= aForceOpValve[29],
	bValveInterlock_In	:= aILK_AV[29] ,		
	bPMCCtrl_In			:= GVL.stPMCtoPLC.aAV[29] ,
	bValveOpen_Out		=> aAV[29] 	
);				
				
AV[30]				
(	bValveEnable_In 	:= TRUE ,		
	bInterlock1_In		:= bEMOStatus ,	
	bInterlock2_In		:= TRUE ,	
	bInterlock3_In		:= TRUE ,	
	bInterlock4_In		:= TRUE ,	
	bInterlock5_In		:= TRUE ,	
	bForceOpen_In		:= aForceOpValve[30],
	bValveInterlock_In	:= aILK_AV[30] ,		
	bPMCCtrl_In			:= GVL.stPMCtoPLC.aAV[30] ,
	bValveOpen_Out		=> aAV[30] 	
);				
				
AV[31]				
(	bValveEnable_In 	:= TRUE ,		
	bInterlock1_In		:= bEMOStatus ,	
	bInterlock2_In		:= TRUE ,	
	bInterlock3_In		:= TRUE ,	
	bInterlock4_In		:= TRUE ,	
	bInterlock5_In		:= TRUE ,	
	bForceOpen_In		:= aForceOpValve[31],
	bValveInterlock_In	:= aILK_AV[31] ,		
	bPMCCtrl_In			:= GVL.stPMCtoPLC.aAV[31] ,
	bValveOpen_Out		=> aAV[31] 	
);				
				
AV[32]				
(	bValveEnable_In 	:= TRUE ,		
	bInterlock1_In		:= bEMOStatus ,	
	bInterlock2_In		:= TRUE ,	
	bInterlock3_In		:= TRUE ,	
	bInterlock4_In		:= TRUE ,	
	bInterlock5_In		:= TRUE ,	
	bForceOpen_In		:= aForceOpValve[32],
	bValveInterlock_In	:= aILK_AV[32] ,		
	bPMCCtrl_In			:= GVL.stPMCtoPLC.aAV[32] ,
	bValveOpen_Out		=> aAV[32] 	
);				
				
AV[33]				
(	bValveEnable_In 	:= TRUE ,		
	bInterlock1_In		:= bEMOStatus ,	
	bInterlock2_In		:= TRUE ,	
	bInterlock3_In		:= TRUE ,	
	bInterlock4_In		:= TRUE ,	
	bInterlock5_In		:= TRUE ,	
	bForceOpen_In		:= aForceOpValve[33],
	bValveInterlock_In	:= aILK_AV[33] ,		
	bPMCCtrl_In			:= GVL.stPMCtoPLC.aAV[33] ,
	bValveOpen_Out		=> aAV[33] 	
);				
				
AV[34]				
(	bValveEnable_In 	:= TRUE ,		
	bInterlock1_In		:= bEMOStatus ,	
	bInterlock2_In		:= TRUE ,	
	bInterlock3_In		:= TRUE ,	
	bInterlock4_In		:= TRUE ,	
	bInterlock5_In		:= TRUE ,	
	bForceOpen_In		:= aForceOpValve[34],
	bValveInterlock_In	:= aILK_AV[34] ,		
	bPMCCtrl_In			:= GVL.stPMCtoPLC.aAV[34] ,
	bValveOpen_Out		=> aAV[34] 	
);				
				
AV[35]				
(	bValveEnable_In 	:= TRUE ,		
	bInterlock1_In		:= bEMOStatus ,	
	bInterlock2_In		:= TRUE ,	
	bInterlock3_In		:= TRUE ,	
	bInterlock4_In		:= TRUE ,	
	bInterlock5_In		:= TRUE ,	
	bForceOpen_In		:= aForceOpValve[35],
	bValveInterlock_In	:= aILK_AV[35] ,		
	bPMCCtrl_In			:= GVL.stPMCtoPLC.aAV[35] ,
	bValveOpen_Out		=> aAV[35] 	
);				
				
AV[36]				
(	bValveEnable_In 	:= TRUE ,		
	bInterlock1_In		:= bEMOStatus ,	
	bInterlock2_In		:= TRUE ,	
	bInterlock3_In		:= TRUE ,	
	bInterlock4_In		:= TRUE ,	
	bInterlock5_In		:= TRUE ,	
	bForceOpen_In		:= aForceOpValve[36],
	bValveInterlock_In	:= aILK_AV[36] ,		
	bPMCCtrl_In			:= GVL.stPMCtoPLC.aAV[36] ,
	bValveOpen_Out		=> aAV[36] 	
);				
				
AV[37]				
(	bValveEnable_In 	:= TRUE ,		
	bInterlock1_In		:= bEMOStatus ,	
	bInterlock2_In		:= TRUE ,	
	bInterlock3_In		:= TRUE ,	
	bInterlock4_In		:= TRUE ,	
	bInterlock5_In		:= TRUE ,	
	bForceOpen_In		:= aForceOpValve[37],
	bValveInterlock_In	:= aILK_AV[37] ,		
	bPMCCtrl_In			:= GVL.stPMCtoPLC.aAV[37] ,
	bValveOpen_Out		=> aAV[37] 	
);				
				
AV[38]				
(	bValveEnable_In 	:= TRUE ,		
	bInterlock1_In		:= bEMOStatus ,	
	bInterlock2_In		:= TRUE ,	
	bInterlock3_In		:= TRUE ,	
	bInterlock4_In		:= TRUE ,	
	bInterlock5_In		:= TRUE ,	
	bForceOpen_In		:= aForceOpValve[38],
	bValveInterlock_In	:= aILK_AV[38] ,		
	bPMCCtrl_In			:= GVL.stPMCtoPLC.aAV[38] ,
	bValveOpen_Out		=> aAV[38] 	
);				
				
AV[39]				
(	bValveEnable_In 	:= TRUE ,		
	bInterlock1_In		:= bEMOStatus ,	
	bInterlock2_In		:= TRUE ,	
	bInterlock3_In		:= TRUE ,	
	bInterlock4_In		:= TRUE ,	
	bInterlock5_In		:= TRUE ,	
	bForceOpen_In		:= aForceOpValve[39],
	bValveInterlock_In	:= aILK_AV[39] ,		
	bPMCCtrl_In			:= GVL.stPMCtoPLC.aAV[39] ,
	bValveOpen_Out		=> aAV[39] 	
);				
				
AV[40]				
(	bValveEnable_In 	:= TRUE ,		
	bInterlock1_In		:= bEMOStatus ,	
	bInterlock2_In		:= TRUE ,	
	bInterlock3_In		:= TRUE ,	
	bInterlock4_In		:= TRUE ,	
	bInterlock5_In		:= TRUE ,	
	bForceOpen_In		:= aForceOpValve[40],
	bValveInterlock_In	:= aILK_AV[40] ,		
	bPMCCtrl_In			:= GVL.stPMCtoPLC.aAV[40] ,
	bValveOpen_Out		=> aAV[40] 	
);				
				
AV[41]				
(	bValveEnable_In 	:= TRUE ,		
	bInterlock1_In		:= bEMOStatus ,	
	bInterlock2_In		:= TRUE ,	
	bInterlock3_In		:= TRUE ,	
	bInterlock4_In		:= TRUE ,	
	bInterlock5_In		:= TRUE ,	
	bForceOpen_In		:= aForceOpValve[41],
	bValveInterlock_In	:= aILK_AV[41] ,		
	bPMCCtrl_In			:= GVL.stPMCtoPLC.aAV[41] ,
	bValveOpen_Out		=> aAV[41] 	
);				
				
AV[42]				
(	bValveEnable_In 	:= TRUE ,		
	bInterlock1_In		:= bEMOStatus ,	
	bInterlock2_In		:= TRUE ,	
	bInterlock3_In		:= TRUE ,	
	bInterlock4_In		:= TRUE ,	
	bInterlock5_In		:= TRUE ,	
	bForceOpen_In		:= aForceOpValve[42],
	bValveInterlock_In	:= aILK_AV[42] ,		
	bPMCCtrl_In			:= GVL.stPMCtoPLC.aAV[42] ,
	bValveOpen_Out		=> aAV[42] 	
);				
				
AV[43]				
(	bValveEnable_In 	:= TRUE ,		
	bInterlock1_In		:= bEMOStatus ,	
	bInterlock2_In		:= TRUE ,	
	bInterlock3_In		:= TRUE ,	
	bInterlock4_In		:= TRUE ,	
	bInterlock5_In		:= TRUE ,	
	bForceOpen_In		:= aForceOpValve[43],
	bValveInterlock_In	:= aILK_AV[43] ,		
	bPMCCtrl_In			:= GVL.stPMCtoPLC.aAV[43] ,
	bValveOpen_Out		=> aAV[43] 	
);				
				
AV[44]				
(	bValveEnable_In 	:= TRUE ,		
	bInterlock1_In		:= bEMOStatus ,	
	bInterlock2_In		:= TRUE ,	
	bInterlock3_In		:= TRUE ,	
	bInterlock4_In		:= TRUE ,	
	bInterlock5_In		:= TRUE ,	
	bForceOpen_In		:= aForceOpValve[44],
	bValveInterlock_In	:= aILK_AV[44] ,		
	bPMCCtrl_In			:= GVL.stPMCtoPLC.aAV[44] ,
	bValveOpen_Out		=> aAV[44] 	
);				
				
AV[45]				
(	bValveEnable_In 	:= TRUE ,		
	bInterlock1_In		:= bEMOStatus ,	
	bInterlock2_In		:= TRUE ,	
	bInterlock3_In		:= TRUE ,	
	bInterlock4_In		:= TRUE ,	
	bInterlock5_In		:= TRUE ,	
	bForceOpen_In		:= aForceOpValve[45],
	bValveInterlock_In	:= aILK_AV[45] ,		
	bPMCCtrl_In			:= GVL.stPMCtoPLC.aAV[45] ,
	bValveOpen_Out		=> aAV[45] 	
);				
				
AV[46]				
(	bValveEnable_In 	:= TRUE ,		
	bInterlock1_In		:= bEMOStatus ,	
	bInterlock2_In		:= TRUE ,	
	bInterlock3_In		:= TRUE ,	
	bInterlock4_In		:= TRUE ,	
	bInterlock5_In		:= TRUE ,	
	bForceOpen_In		:= aForceOpValve[46],
	bValveInterlock_In	:= aILK_AV[46] ,		
	bPMCCtrl_In			:= GVL.stPMCtoPLC.aAV[46] ,
	bValveOpen_Out		=> aAV[46] 	
);				
				
AV[47]				
(	bValveEnable_In 	:= TRUE ,		
	bInterlock1_In		:= bEMOStatus ,	
	bInterlock2_In		:= TRUE ,	
	bInterlock3_In		:= TRUE ,	
	bInterlock4_In		:= TRUE ,	
	bInterlock5_In		:= TRUE ,	
	bForceOpen_In		:= aForceOpValve[47],
	bValveInterlock_In	:= aILK_AV[47] ,		
	bPMCCtrl_In			:= GVL.stPMCtoPLC.aAV[47] ,
	bValveOpen_Out		=> aAV[47] 	
);				
				
AV[48]				
(	bValveEnable_In 	:= TRUE ,		
	bInterlock1_In		:= bEMOStatus ,	
	bInterlock2_In		:= TRUE ,	
	bInterlock3_In		:= TRUE ,	
	bInterlock4_In		:= TRUE ,	
	bInterlock5_In		:= TRUE ,	
	bForceOpen_In		:= aForceOpValve[48],
	bValveInterlock_In	:= aILK_AV[48] ,		
	bPMCCtrl_In			:= GVL.stPMCtoPLC.aAV[48] ,
	bValveOpen_Out		=> aAV[48] 	
);				
				
AV[49]				
(	bValveEnable_In 	:= TRUE ,		
	bInterlock1_In		:= bEMOStatus ,	
	bInterlock2_In		:= TRUE ,	
	bInterlock3_In		:= TRUE ,	
	bInterlock4_In		:= TRUE ,	
	bInterlock5_In		:= TRUE ,	
	bForceOpen_In		:= aForceOpValve[49],
	bValveInterlock_In	:= aILK_AV[49] ,		
	bPMCCtrl_In			:= GVL.stPMCtoPLC.aAV[49] ,
	bValveOpen_Out		=> aAV[49] 	
);				
				
AV[50]				
(	bValveEnable_In 	:= TRUE ,		
	bInterlock1_In		:= bEMOStatus ,	
	bInterlock2_In		:= TRUE ,	
	bInterlock3_In		:= TRUE ,	
	bInterlock4_In		:= TRUE ,	
	bInterlock5_In		:= TRUE ,	
	bForceOpen_In		:= aForceOpValve[50],
	bValveInterlock_In	:= aILK_AV[50] ,		
	bPMCCtrl_In			:= GVL.stPMCtoPLC.aAV[50] ,
	bValveOpen_Out		=> aAV[50] 	
);				
				
AV[51]				
(	bValveEnable_In 	:= TRUE ,		
	bInterlock1_In		:= bEMOStatus ,	
	bInterlock2_In		:= TRUE ,	
	bInterlock3_In		:= TRUE ,	
	bInterlock4_In		:= TRUE ,	
	bInterlock5_In		:= TRUE ,	
	bForceOpen_In		:= aForceOpValve[51],
	bValveInterlock_In	:= aILK_AV[51] ,		
	bPMCCtrl_In			:= GVL.stPMCtoPLC.aAV[51] ,
	bValveOpen_Out		=> aAV[51] 	
);				
				
AV[52]				
(	bValveEnable_In 	:= TRUE ,		
	bInterlock1_In		:= bEMOStatus ,	
	bInterlock2_In		:= TRUE ,	
	bInterlock3_In		:= TRUE ,	
	bInterlock4_In		:= TRUE ,	
	bInterlock5_In		:= TRUE ,	
	bForceOpen_In		:= aForceOpValve[52],
	bValveInterlock_In	:= aILK_AV[52] ,		
	bPMCCtrl_In			:= GVL.stPMCtoPLC.aAV[52] ,
	bValveOpen_Out		=> aAV[52] 	
);				
				
AV[53]				
(	bValveEnable_In 	:= TRUE ,		
	bInterlock1_In		:= bEMOStatus ,	
	bInterlock2_In		:= TRUE ,	
	bInterlock3_In		:= TRUE ,	
	bInterlock4_In		:= TRUE ,	
	bInterlock5_In		:= TRUE ,	
	bForceOpen_In		:= aForceOpValve[53],
	bValveInterlock_In	:= aILK_AV[53] ,		
	bPMCCtrl_In			:= GVL.stPMCtoPLC.aAV[53] ,
	bValveOpen_Out		=> aAV[53] 	
);				
				
AV[54]				
(	bValveEnable_In 	:= TRUE ,		
	bInterlock1_In		:= bEMOStatus ,	
	bInterlock2_In		:= TRUE ,	
	bInterlock3_In		:= TRUE ,	
	bInterlock4_In		:= TRUE ,	
	bInterlock5_In		:= TRUE ,	
	bForceOpen_In		:= aForceOpValve[54],
	bValveInterlock_In	:= aILK_AV[54] ,		
	bPMCCtrl_In			:= GVL.stPMCtoPLC.aAV[54] ,
	bValveOpen_Out		=> aAV[54] 	
);				
				
AV[55]				
(	bValveEnable_In 	:= TRUE ,		
	bInterlock1_In		:= bEMOStatus ,	
	bInterlock2_In		:= TRUE ,	
	bInterlock3_In		:= TRUE ,	
	bInterlock4_In		:= TRUE ,	
	bInterlock5_In		:= TRUE ,	
	bForceOpen_In		:= aForceOpValve[55],
	bValveInterlock_In	:= aILK_AV[55] ,		
	bPMCCtrl_In			:= GVL.stPMCtoPLC.aAV[55] ,
	bValveOpen_Out		=> aAV[55] 	
);				
				
AV[56]				
(	bValveEnable_In 	:= TRUE ,		
	bInterlock1_In		:= bEMOStatus ,	
	bInterlock2_In		:= TRUE ,	
	bInterlock3_In		:= TRUE ,	
	bInterlock4_In		:= TRUE ,	
	bInterlock5_In		:= TRUE ,	
	bForceOpen_In		:= aForceOpValve[56],
	bValveInterlock_In	:= aILK_AV[56] ,		
	bPMCCtrl_In			:= GVL.stPMCtoPLC.aAV[56] ,
	bValveOpen_Out		=> aAV[56] 	
);				
				
AV[57]				
(	bValveEnable_In 	:= TRUE ,		
	bInterlock1_In		:= bEMOStatus ,	
	bInterlock2_In		:= TRUE ,	
	bInterlock3_In		:= TRUE ,	
	bInterlock4_In		:= TRUE ,	
	bInterlock5_In		:= TRUE ,	
	bForceOpen_In		:= aForceOpValve[57],
	bValveInterlock_In	:= aILK_AV[57] ,		
	bPMCCtrl_In			:= GVL.stPMCtoPLC.aAV[57] ,
	bValveOpen_Out		=> aAV[57] 	
);				
				
AV[58]				
(	bValveEnable_In 	:= TRUE ,		
	bInterlock1_In		:= bEMOStatus ,	
	bInterlock2_In		:= TRUE ,	
	bInterlock3_In		:= TRUE ,	
	bInterlock4_In		:= TRUE ,	
	bInterlock5_In		:= TRUE ,
	bForceOpen_In		:= aForceOpValve[58],	
	bValveInterlock_In	:= aILK_AV[58] ,		
	bPMCCtrl_In			:= GVL.stPMCtoPLC.aAV[58] ,
	bValveOpen_Out		=> aAV[58] 	
);				
				
AV[59]				
(	bValveEnable_In 	:= TRUE ,		
	bInterlock1_In		:= bEMOStatus ,	
	bInterlock2_In		:= TRUE ,	
	bInterlock3_In		:= TRUE ,	
	bInterlock4_In		:= TRUE ,	
	bInterlock5_In		:= TRUE ,	
	bForceOpen_In		:= aForceOpValve[59],
	bValveInterlock_In	:= aILK_AV[59] ,		
	bPMCCtrl_In			:= GVL.stPMCtoPLC.aAV[59] ,
	bValveOpen_Out		=> aAV[59] 	
);				
				
AV[60]	//auto valve				
(	bValveEnable_In 	:= TRUE ,		
	bInterlock1_In		:= bEMOStatus ,	
	bInterlock2_In		:= TRUE ,	
	bInterlock3_In		:= TRUE ,	
	bInterlock4_In		:= TRUE ,	
	bInterlock5_In		:= TRUE ,	
	bForceOpen_In		:= aForceOpValve[60],
	bValveInterlock_In	:= aILK_AV[60] ,		
	bPMCCtrl_In			:= TRUE(*GVL.stPMCtoPLC.aAV[60]*) ,
	bValveOpen_Out		=> aAV[60] 	
);				
				
AV[61]				
(	bValveEnable_In 	:= TRUE ,		
	bInterlock1_In		:= bEMOStatus ,	
	bInterlock2_In		:= TRUE ,	
	bInterlock3_In		:= TRUE ,	
	bInterlock4_In		:= TRUE ,	
	bInterlock5_In		:= TRUE ,	
	bForceOpen_In		:= aForceOpValve[61],
	bValveInterlock_In	:= aILK_AV[61] ,		
	bPMCCtrl_In			:= GVL.stPMCtoPLC.aAV[61] ,
	bValveOpen_Out		=> aAV[61] 	
);				
				
AV[62]				
(	bValveEnable_In 	:= TRUE ,		
	bInterlock1_In		:= bEMOStatus ,	
	bInterlock2_In		:= TRUE ,	
	bInterlock3_In		:= TRUE ,	
	bInterlock4_In		:= TRUE ,	
	bInterlock5_In		:= TRUE ,	
	bForceOpen_In		:= aForceOpValve[62],
	bValveInterlock_In	:= aILK_AV[62] ,		
	bPMCCtrl_In			:= GVL.stPMCtoPLC.aAV[62] ,
	bValveOpen_Out		=> aAV[62] 	
);				
				
AV[63]				
(	bValveEnable_In 	:= TRUE ,		
	bInterlock1_In		:= bEMOStatus ,	
	bInterlock2_In		:= TRUE ,	
	bInterlock3_In		:= TRUE ,	
	bInterlock4_In		:= TRUE ,	
	bInterlock5_In		:= TRUE ,	
	bForceOpen_In		:= aForceOpValve[63],
	bValveInterlock_In	:= aILK_AV[63] ,		
	bPMCCtrl_In			:= GVL.stPMCtoPLC.aAV[63] ,
	bValveOpen_Out		=> aAV[63] 	
);				
				
AV[64]				
(	bValveEnable_In 	:= TRUE ,		
	bInterlock1_In		:= bEMOStatus ,	
	bInterlock2_In		:= TRUE ,	
	bInterlock3_In		:= TRUE ,	
	bInterlock4_In		:= TRUE ,	
	bInterlock5_In		:= TRUE ,	
	bForceOpen_In		:= aForceOpValve[64],
	bValveInterlock_In	:= aILK_AV[64] ,		
	bPMCCtrl_In			:= GVL.stPMCtoPLC.aAV[64] ,
	bValveOpen_Out		=> aAV[64] 	
);				
				
(*AV[65]				
(	bValveEnable_In 	:= TRUE ,		
	bInterlock1_In		:= bEMOStatus ,	
	bInterlock2_In		:= TRUE ,	
	bInterlock3_In		:= TRUE ,	
	bInterlock4_In		:= TRUE ,	
	bInterlock5_In		:= TRUE ,
	bForceOpen_In		:= aForceOpValve[65],	
	bValveInterlock_In	:= aILK_AV[65] ,		
	bPMCCtrl_In			:= GVL.stPMCtoPLC.aAV[65] ,
	bValveOpen_Out		=> aAV[65] 	
);	*)	

AV65Open				
(	bValveEnable_In 	:= TRUE ,		
	bInterlock1_In		:= bEMOStatus ,	
	bInterlock2_In		:= TRUE ,	
	bInterlock3_In		:= TRUE ,	
	bInterlock4_In		:= TRUE ,	
	bInterlock5_In		:= TRUE ,
	bForceOpen_In		:= bForceAV65Open,	
	bValveInterlock_In	:= aILK_AV[65] ,		
	bPMCCtrl_In			:= GVL.stPMCtoPLC.bAV65Open ,
	bValveOpen_Out		=> GVL.bAV65Open 	
);	

AV65Close				
(	bValveEnable_In 	:= TRUE ,		
	bInterlock1_In		:= bEMOStatus ,	
	bInterlock2_In		:= TRUE ,	
	bInterlock3_In		:= TRUE ,	
	bInterlock4_In		:= TRUE ,	
	bInterlock5_In		:= TRUE ,
	bForceOpen_In		:= bForceAV65Close,	
	bValveInterlock_In	:= aILK_AV[65] ,		
	bPMCCtrl_In			:= GVL.stPMCtoPLC.bAV65Close ,
	bValveOpen_Out		=> GVL.bAV65Close 	
);	
				
AV[66]				
(	bValveEnable_In 	:= TRUE ,		
	bInterlock1_In		:= bEMOStatus ,	
	bInterlock2_In		:= TRUE ,	
	bInterlock3_In		:= TRUE ,	
	bInterlock4_In		:= TRUE ,	
	bInterlock5_In		:= TRUE ,	
	bForceOpen_In		:= aForceOpValve[66],
	bValveInterlock_In	:= aILK_AV[66] ,		
	bPMCCtrl_In			:= GVL.stPMCtoPLC.aAV[66] ,
	bValveOpen_Out		=> aAV[66] 	
);				
				
AV[67]				
(	bValveEnable_In 	:= TRUE ,		
	bInterlock1_In		:= bEMOStatus ,	
	bInterlock2_In		:= TRUE ,	
	bInterlock3_In		:= TRUE ,	
	bInterlock4_In		:= TRUE ,	
	bInterlock5_In		:= TRUE ,	
	bForceOpen_In		:= aForceOpValve[67],
	bValveInterlock_In	:= aILK_AV[67] ,		
	bPMCCtrl_In			:= GVL.stPMCtoPLC.aAV[67] ,
	bValveOpen_Out		=> aAV[67] 	
);				
				
AV[68]	// auto valve				
(	bValveEnable_In 	:= TRUE ,		
	bInterlock1_In		:= bEMOStatus ,	
	bInterlock2_In		:= TRUE ,	
	bInterlock3_In		:= TRUE ,	
	bInterlock4_In		:= TRUE ,	
	bInterlock5_In		:= TRUE ,	
	bForceOpen_In		:= aForceOpValve[68],
	bValveInterlock_In	:= aILK_AV[68] ,		
	bPMCCtrl_In			:= TRUE(*GVL.stPMCtoPLC.aAV[68]*) ,
	bValveOpen_Out		=> aAV[68] 	
);				
				
AV[69]				
(	bValveEnable_In 	:= TRUE ,		
	bInterlock1_In		:= bEMOStatus ,	
	bInterlock2_In		:= TRUE ,	
	bInterlock3_In		:= TRUE ,	
	bInterlock4_In		:= TRUE ,	
	bInterlock5_In		:= TRUE ,	
	bForceOpen_In		:= aForceOpValve[69],
	bValveInterlock_In	:= aILK_AV[69] ,		
	bPMCCtrl_In			:= GVL.stPMCtoPLC.aAV[69] ,
	bValveOpen_Out		=> aAV[69] 	
);				
				
AV[70]				
(	bValveEnable_In 	:= TRUE ,		
	bInterlock1_In		:= bEMOStatus ,	
	bInterlock2_In		:= TRUE ,	
	bInterlock3_In		:= TRUE ,	
	bInterlock4_In		:= TRUE ,	
	bInterlock5_In		:= TRUE ,	
	bForceOpen_In		:= aForceOpValve[70],
	bValveInterlock_In	:= aILK_AV[70] ,		
	bPMCCtrl_In			:= GVL.stPMCtoPLC.aAV[70] ,
	bValveOpen_Out		=> aAV[70] 	
);				
				
AV[71]				
(	bValveEnable_In 	:= TRUE ,		
	bInterlock1_In		:= bEMOStatus ,	
	bInterlock2_In		:= TRUE ,	
	bInterlock3_In		:= TRUE ,	
	bInterlock4_In		:= TRUE ,	
	bInterlock5_In		:= TRUE ,	
	bForceOpen_In		:= aForceOpValve[71],
	bValveInterlock_In	:= aILK_AV[71] ,		
	bPMCCtrl_In			:= GVL.stPMCtoPLC.aAV[71] ,
	bValveOpen_Out		=> aAV[71] 	
);				
				
AV[72]				
(	bValveEnable_In 	:= TRUE ,		
	bInterlock1_In		:= bEMOStatus ,	
	bInterlock2_In		:= TRUE ,	
	bInterlock3_In		:= TRUE ,	
	bInterlock4_In		:= TRUE ,	
	bInterlock5_In		:= TRUE ,	
	bForceOpen_In		:= aForceOpValve[72],
	bValveInterlock_In	:= aILK_AV[72] ,		
	bPMCCtrl_In			:= GVL.stPMCtoPLC.aAV[72] ,
	bValveOpen_Out		=> aAV[72] 	
);				
				
AV[73]	// auto valve				
(	bValveEnable_In 	:= TRUE ,		
	bInterlock1_In		:= bEMOStatus ,	
	bInterlock2_In		:= TRUE ,	
	bInterlock3_In		:= TRUE ,	
	bInterlock4_In		:= TRUE ,	
	bInterlock5_In		:= TRUE ,	
	bForceOpen_In		:= aForceOpValve[73],
	bValveInterlock_In	:= aILK_AV[73] ,		
	bPMCCtrl_In			:= TRUE(*GVL.stPMCtoPLC.aAV[73]*) ,
	bValveOpen_Out		=> aAV[73] 	
);				
				
AV[74]	// auto valve				
(	bValveEnable_In 	:= TRUE ,		
	bInterlock1_In		:= bEMOStatus ,	
	bInterlock2_In		:= TRUE ,	
	bInterlock3_In		:= TRUE ,	
	bInterlock4_In		:= TRUE ,	
	bInterlock5_In		:= TRUE ,	
	bForceOpen_In		:= aForceOpValve[74],
	bValveInterlock_In	:= aILK_AV[74] ,		
	bPMCCtrl_In			:= TRUE(*GVL.stPMCtoPLC.aAV[74]*) ,
	bValveOpen_Out		=> aAV[74] 	
);				
				
AV[75]				
(	bValveEnable_In 	:= TRUE ,		
	bInterlock1_In		:= bEMOStatus ,	
	bInterlock2_In		:= TRUE ,	
	bInterlock3_In		:= TRUE ,	
	bInterlock4_In		:= TRUE ,	
	bInterlock5_In		:= TRUE ,	
	bForceOpen_In		:= aForceOpValve[75],
	bValveInterlock_In	:= aILK_AV[75] ,		
	bPMCCtrl_In			:= GVL.stPMCtoPLC.aAV[75] ,
	bValveOpen_Out		=> aAV[75] 	
);				
				
AV[76]				
(	bValveEnable_In 	:= TRUE ,		
	bInterlock1_In		:= bEMOStatus ,	
	bInterlock2_In		:= TRUE ,	
	bInterlock3_In		:= TRUE ,	
	bInterlock4_In		:= TRUE ,	
	bInterlock5_In		:= TRUE ,	
	bForceOpen_In		:= aForceOpValve[76],
	bValveInterlock_In	:= aILK_AV[76] ,		
	bPMCCtrl_In			:= GVL.stPMCtoPLC.aAV[76] ,
	bValveOpen_Out		=> aAV[76] 	
);				
				
AV[77]				
(	bValveEnable_In 	:= TRUE ,		
	bInterlock1_In		:= bEMOStatus ,	
	bInterlock2_In		:= TRUE ,	
	bInterlock3_In		:= TRUE ,	
	bInterlock4_In		:= TRUE ,	
	bInterlock5_In		:= TRUE ,	
	bForceOpen_In		:= aForceOpValve[77],
	bValveInterlock_In	:= aILK_AV[77] ,		
	bPMCCtrl_In			:= TRUE(*GVL.stPMCtoPLC.aAV[77]*) ,
	bValveOpen_Out		=> aAV[77] 	
);				
				
AV[78]				
(	bValveEnable_In 	:= TRUE ,		
	bInterlock1_In		:= bEMOStatus ,	
	bInterlock2_In		:= TRUE ,	
	bInterlock3_In		:= TRUE ,	
	bInterlock4_In		:= TRUE ,	
	bInterlock5_In		:= TRUE ,	
	bForceOpen_In		:= aForceOpValve[78],
	bValveInterlock_In	:= aILK_AV[78] ,		
	bPMCCtrl_In			:= GVL.stPMCtoPLC.aAV[78] ,
	bValveOpen_Out		=> aAV[78] 	
);		
		
AV79Open				
(	bValveEnable_In 	:= TRUE ,		
	bInterlock1_In		:= bEMOStatus ,	
	bInterlock2_In		:= TRUE ,	
	bInterlock3_In		:= TRUE ,	
	bInterlock4_In		:= TRUE ,	
	bInterlock5_In		:= TRUE ,
	bForceOpen_In		:= bForceAV79Open,	
	bValveInterlock_In	:= aILK_AV[79] ,		
	bPMCCtrl_In			:= GVL.stPMCtoPLC.bAV79Open ,
	bValveOpen_Out		=> GVL.bAV79Open 	
);	

AV79Close				
(	bValveEnable_In 	:= TRUE ,		
	bInterlock1_In		:= bEMOStatus ,	
	bInterlock2_In		:= TRUE ,	
	bInterlock3_In		:= TRUE ,	
	bInterlock4_In		:= TRUE ,	
	bInterlock5_In		:= TRUE ,
	bForceOpen_In		:= bForceAV79Close,	
	bValveInterlock_In	:= aILK_AV[79] ,		
	bPMCCtrl_In			:= GVL.stPMCtoPLC.bAV79Close ,
	bValveOpen_Out		=> GVL.bAV79Close 	
);
		
(*AV[79]				
(	bValveEnable_In 	:= TRUE ,		
	bInterlock1_In		:= bEMOStatus ,	
	bInterlock2_In		:= TRUE ,	
	bInterlock3_In		:= TRUE ,	
	bInterlock4_In		:= TRUE ,	
	bInterlock5_In		:= TRUE ,	
	bForceOpen_In		:= aForceOpValve[79],
	bValveInterlock_In	:= aILK_AV[79] ,		
	bPMCCtrl_In			:= GVL.stPMCtoPLC.aAV[79] ,
	bValveOpen_Out		=> aAV[79] 	
);	*)			
				
AV[80]				
(	bValveEnable_In 	:= TRUE ,		
	bInterlock1_In		:= bEMOStatus ,	
	bInterlock2_In		:= TRUE ,	
	bInterlock3_In		:= TRUE ,	
	bInterlock4_In		:= TRUE ,	
	bInterlock5_In		:= TRUE ,	
	bForceOpen_In		:= aForceOpValve[80],
	bValveInterlock_In	:= aILK_AV[80] ,		
	bPMCCtrl_In			:= GVL.stPMCtoPLC.aAV[80] ,
	bValveOpen_Out		=> aAV[80] 	
);				
				
AV[81]				
(	bValveEnable_In 	:= TRUE ,		
	bInterlock1_In		:= bEMOStatus ,	
	bInterlock2_In		:= TRUE ,	
	bInterlock3_In		:= TRUE ,	
	bInterlock4_In		:= TRUE ,	
	bInterlock5_In		:= TRUE ,	
	bForceOpen_In		:= aForceOpValve[81],
	bValveInterlock_In	:= aILK_AV[81] ,		
	bPMCCtrl_In			:= GVL.stPMCtoPLC.aAV[81] ,
	bValveOpen_Out		=> aAV[81] 	
);				
				
AV[82]				
(	bValveEnable_In 	:= TRUE ,		
	bInterlock1_In		:= bEMOStatus ,	
	bInterlock2_In		:= TRUE ,	
	bInterlock3_In		:= TRUE ,	
	bInterlock4_In		:= TRUE ,	
	bInterlock5_In		:= TRUE ,	
	bForceOpen_In		:= aForceOpValve[82],
	bValveInterlock_In	:= aILK_AV[82] ,		
	bPMCCtrl_In			:= GVL.stPMCtoPLC.aAV[82] ,
	bValveOpen_Out		=> aAV[82] 	
);				
				
AV[83]				
(	bValveEnable_In 	:= TRUE ,		
	bInterlock1_In		:= bEMOStatus ,	
	bInterlock2_In		:= TRUE ,	
	bInterlock3_In		:= TRUE ,	
	bInterlock4_In		:= TRUE ,	
	bInterlock5_In		:= TRUE ,	
	bForceOpen_In		:= aForceOpValve[83],
	bValveInterlock_In	:= aILK_AV[83] ,		
	bPMCCtrl_In			:= GVL.stPMCtoPLC.aAV[83] ,
	bValveOpen_Out		=> aAV[83] 	
);				
				
AV[84]				
(	bValveEnable_In 	:= TRUE ,		
	bInterlock1_In		:= bEMOStatus ,	
	bInterlock2_In		:= TRUE ,	
	bInterlock3_In		:= TRUE ,	
	bInterlock4_In		:= TRUE ,	
	bInterlock5_In		:= TRUE ,	
	bForceOpen_In		:= aForceOpValve[84],
	bValveInterlock_In	:= aILK_AV[84] ,		
	bPMCCtrl_In			:= GVL.stPMCtoPLC.aAV[84] ,
	bValveOpen_Out		=> aAV[84] 	
);				
				
AV[85]				
(	bValveEnable_In 	:= TRUE ,		
	bInterlock1_In		:= bEMOStatus ,	
	bInterlock2_In		:= TRUE ,	
	bInterlock3_In		:= TRUE ,	
	bInterlock4_In		:= TRUE ,	
	bInterlock5_In		:= TRUE ,	
	bForceOpen_In		:= aForceOpValve[85],
	bValveInterlock_In	:= aILK_AV[85] ,		
	bPMCCtrl_In			:= GVL.stPMCtoPLC.aAV[85] ,
	bValveOpen_Out		=> aAV[85] 	
);				
				
AV[86]				
(	bValveEnable_In 	:= TRUE ,		
	bInterlock1_In		:= bEMOStatus ,	
	bInterlock2_In		:= TRUE ,	
	bInterlock3_In		:= TRUE ,	
	bInterlock4_In		:= TRUE ,	
	bInterlock5_In		:= TRUE ,	
	bForceOpen_In		:= aForceOpValve[86],
	bValveInterlock_In	:= aILK_AV[86] ,		
	bPMCCtrl_In			:= GVL.stPMCtoPLC.aAV[86] ,
	bValveOpen_Out		=> aAV[86] 	
);				
				
AV[87]				
(	bValveEnable_In 	:= TRUE ,		
	bInterlock1_In		:= bEMOStatus ,	
	bInterlock2_In		:= TRUE ,	
	bInterlock3_In		:= TRUE ,	
	bInterlock4_In		:= TRUE ,	
	bInterlock5_In		:= TRUE ,	
	bForceOpen_In		:= aForceOpValve[87],
	bValveInterlock_In	:= aILK_AV[87] ,		
	bPMCCtrl_In			:= GVL.stPMCtoPLC.aAV[87] ,
	bValveOpen_Out		=> aAV[87] 	
);				
				
AV[88]				
(	bValveEnable_In 	:= TRUE ,		
	bInterlock1_In		:= bEMOStatus ,	
	bInterlock2_In		:= TRUE ,	
	bInterlock3_In		:= TRUE ,	
	bInterlock4_In		:= TRUE ,	
	bInterlock5_In		:= TRUE ,	
	bForceOpen_In		:= aForceOpValve[88],
	bValveInterlock_In	:= aILK_AV[88] ,		
	bPMCCtrl_In			:= GVL.stPMCtoPLC.aAV[88] ,
	bValveOpen_Out		=> aAV[88] 	
);				
				
AV[89]				
(	bValveEnable_In 	:= TRUE ,		
	bInterlock1_In		:= bEMOStatus ,	
	bInterlock2_In		:= TRUE ,	
	bInterlock3_In		:= TRUE ,	
	bInterlock4_In		:= TRUE ,	
	bInterlock5_In		:= TRUE ,	
	bForceOpen_In		:= aForceOpValve[89],
	bValveInterlock_In	:= aILK_AV[89] ,		
	bPMCCtrl_In			:= GVL.stPMCtoPLC.aAV[89] ,
	bValveOpen_Out		=> aAV[89] 	
);				
				
AV[90]				
(	bValveEnable_In 	:= TRUE ,		
	bInterlock1_In		:= bEMOStatus ,	
	bInterlock2_In		:= TRUE ,	
	bInterlock3_In		:= TRUE ,	
	bInterlock4_In		:= TRUE ,	
	bInterlock5_In		:= TRUE ,	
	bForceOpen_In		:= aForceOpValve[90],
	bValveInterlock_In	:= aILK_AV[90] ,		
	bPMCCtrl_In			:= GVL.stPMCtoPLC.aAV[90] ,
	bValveOpen_Out		=> aAV[90] 	
);				
				
(*AV[91]				
(	bValveEnable_In 	:= TRUE ,		
	bInterlock1_In		:= bEMOStatus ,	
	bInterlock2_In		:= TRUE ,	
	bInterlock3_In		:= TRUE ,	
	bInterlock4_In		:= TRUE ,	
	bInterlock5_In		:= TRUE ,	
	bForceOpen_In		:= aForceOpValve[91],
	bValveInterlock_In	:= aILK_AV[91] ,		
	bPMCCtrl_In			:= FALSE ,
	bValveOpen_Out		=> aAV[91] 	
);	*)

AV91Open				
(	bValveEnable_In 	:= TRUE ,		
	bInterlock1_In		:= bEMOStatus ,	
	bInterlock2_In		:= TRUE ,	
	bInterlock3_In		:= TRUE ,	
	bInterlock4_In		:= TRUE ,	
	bInterlock5_In		:= TRUE ,
	bForceOpen_In		:= bForceAV91Open,	
	bValveInterlock_In	:= TRUE(*aILK_AV[91]*) ,		
	bPMCCtrl_In			:= GVL.stPMCtoPLC.bAV91Open ,
	bValveOpen_Out		=> GVL.bAV91Open 	
);	

AV91Close				
(	bValveEnable_In 	:= TRUE ,		
	bInterlock1_In		:= bEMOStatus ,	
	bInterlock2_In		:= TRUE ,	
	bInterlock3_In		:= TRUE ,	
	bInterlock4_In		:= TRUE ,	
	bInterlock5_In		:= TRUE ,
	bForceOpen_In		:= bForceAV91Close,	
	bValveInterlock_In	:= TRUE(*aILK_AV[91]*) ,		
	bPMCCtrl_In			:= GVL.stPMCtoPLC.bAV91Close ,
	bValveOpen_Out		=> GVL.bAV91Close 	
);			
				
AV[92]				
(	bValveEnable_In 	:= TRUE ,		
	bInterlock1_In		:= bEMOStatus ,	
	bInterlock2_In		:= TRUE ,	
	bInterlock3_In		:= TRUE ,	
	bInterlock4_In		:= TRUE ,	
	bInterlock5_In		:= TRUE ,	
	bForceOpen_In		:= aForceOpValve[92],
	bValveInterlock_In	:= aILK_AV[92] ,		
	bPMCCtrl_In			:= TRUE ,
	bValveOpen_Out		=> aAV[92] 	
);				
				
AV[93]				
(	bValveEnable_In 	:= TRUE ,		
	bInterlock1_In		:= bEMOStatus ,	
	bInterlock2_In		:= TRUE ,	
	bInterlock3_In		:= TRUE ,	
	bInterlock4_In		:= TRUE ,	
	bInterlock5_In		:= TRUE ,	
	bForceOpen_In		:= aForceOpValve[93],
	bValveInterlock_In	:= aILK_AV[93] ,		
	bPMCCtrl_In			:= GVL.stPMCtoPLC.aAV[93] ,
	bValveOpen_Out		=> aAV[93] 	
);				
				
AV[94]				
(	bValveEnable_In 	:= TRUE ,		
	bInterlock1_In		:= bEMOStatus ,	
	bInterlock2_In		:= TRUE ,	
	bInterlock3_In		:= TRUE ,	
	bInterlock4_In		:= TRUE ,	
	bInterlock5_In		:= TRUE ,
bForceOpen_In		:= aForceOpValve[94],	
	bValveInterlock_In	:= aILK_AV[94] ,		
	bPMCCtrl_In			:= GVL.stPMCtoPLC.aAV[94] ,
	bValveOpen_Out		=> aAV[94] 	
);				
				
AV[95]				
(	bValveEnable_In 	:= TRUE ,		
	bInterlock1_In		:= bEMOStatus ,	
	bInterlock2_In		:= TRUE ,	
	bInterlock3_In		:= TRUE ,	
	bInterlock4_In		:= TRUE ,	
	bInterlock5_In		:= TRUE ,	
	bForceOpen_In		:= aForceOpValve[95],
	bValveInterlock_In	:= aILK_AV[95] ,		
	bPMCCtrl_In			:= GVL.stPMCtoPLC.aAV[95] ,
	bValveOpen_Out		=> aAV[95] 	
);				
				
AV[96]				
(	bValveEnable_In 	:= TRUE ,		
	bInterlock1_In		:= bEMOStatus ,	
	bInterlock2_In		:= TRUE ,	
	bInterlock3_In		:= TRUE ,	
	bInterlock4_In		:= TRUE ,	
	bInterlock5_In		:= TRUE ,	
	bForceOpen_In		:= aForceOpValve[96],
	bValveInterlock_In	:= aILK_AV[96] ,		
	bPMCCtrl_In			:= GVL.stPMCtoPLC.aAV[96] ,
	bValveOpen_Out		=> aAV[96] 	
);				
				
AV[97]				
(	bValveEnable_In 	:= TRUE ,		
	bInterlock1_In		:= bEMOStatus ,	
	bInterlock2_In		:= TRUE ,	
	bInterlock3_In		:= TRUE ,	
	bInterlock4_In		:= TRUE ,	
	bInterlock5_In		:= TRUE ,	
	bForceOpen_In		:= aForceOpValve[97],
	bValveInterlock_In	:= aILK_AV[97] ,		
	bPMCCtrl_In			:= GVL.stPMCtoPLC.aAV[97] ,
	bValveOpen_Out		=> aAV[97] 	
);				
				
AV[98]				
(	bValveEnable_In 	:= TRUE ,		
	bInterlock1_In		:= bEMOStatus ,	
	bInterlock2_In		:= TRUE ,	
	bInterlock3_In		:= TRUE ,	
	bInterlock4_In		:= TRUE ,	
	bInterlock5_In		:= TRUE ,	
	bForceOpen_In		:= aForceOpValve[98],
	bValveInterlock_In	:= aILK_AV[98] ,		
	bPMCCtrl_In			:= GVL.stPMCtoPLC.aAV[98] ,
	bValveOpen_Out		=> aAV[98] 	
);				
				
AV[99]				
(	bValveEnable_In 	:= TRUE ,		
	bInterlock1_In		:= bEMOStatus ,	
	bInterlock2_In		:= TRUE ,	
	bInterlock3_In		:= TRUE ,	
	bInterlock4_In		:= TRUE ,	
	bInterlock5_In		:= TRUE ,	
	bForceOpen_In		:= aForceOpValve[99],
	bValveInterlock_In	:= aILK_AV[99] ,		
	bPMCCtrl_In			:= GVL.stPMCtoPLC.aAV[99] ,
	bValveOpen_Out		=> aAV[99] 	
);				
				
AV[100]				
(	bValveEnable_In 	:= TRUE ,		
	bInterlock1_In		:= bEMOStatus ,	
	bInterlock2_In		:= TRUE ,	
	bInterlock3_In		:= TRUE ,	
	bInterlock4_In		:= TRUE ,	
	bInterlock5_In		:= TRUE ,	
	bForceOpen_In		:= aForceOpValve[100],
	bValveInterlock_In	:= aILK_AV[100] ,		
	bPMCCtrl_In			:= NOT GVL.stPMCtoPLC.T_MNT_sw OR ( GVL.stPMCtoPLC.T_MNT_sw AND GVL.stPMCtoPLC.T_REF_sw AND GVL.stPMCtoPLC.aAV[100] )(*GVL.stPMCtoPLC.aAV[100]*) ,
	bValveOpen_Out		=> aAV[100] 	
);				
				
AV[101]				
(	bValveEnable_In 	:= TRUE ,		
	bInterlock1_In		:= bEMOStatus ,	
	bInterlock2_In		:= TRUE ,	
	bInterlock3_In		:= TRUE ,	
	bInterlock4_In		:= TRUE ,	
	bInterlock5_In		:= TRUE ,	
	bForceOpen_In		:= aForceOpValve[101],
	bValveInterlock_In	:= aILK_AV[101] ,		
	bPMCCtrl_In			:= NOT GVL.stPMCtoPLC.T_MNT_sw OR ( GVL.stPMCtoPLC.T_MNT_sw AND GVL.stPMCtoPLC.T_REF_sw AND GVL.stPMCtoPLC.aAV[101] )(*GVL.stPMCtoPLC.aAV[101]*) ,
	bValveOpen_Out		=> aAV[101] 	
);				
				
AV[102]				
(	bValveEnable_In 	:= TRUE ,		
	bInterlock1_In		:= bEMOStatus ,	
	bInterlock2_In		:= TRUE ,	
	bInterlock3_In		:= TRUE ,	
	bInterlock4_In		:= TRUE ,	
	bInterlock5_In		:= TRUE ,	
	bForceOpen_In		:= aForceOpValve[102],
	bValveInterlock_In	:= aILK_AV[102] ,		
	bPMCCtrl_In			:= GVL.stPMCtoPLC.aAV[102] ,
	bValveOpen_Out		=> aAV[102] 	
);				
				
AV[103]				
(	bValveEnable_In 	:= TRUE ,		
	bInterlock1_In		:= bEMOStatus ,	
	bInterlock2_In		:= TRUE ,	
	bInterlock3_In		:= TRUE ,	
	bInterlock4_In		:= TRUE ,	
	bInterlock5_In		:= TRUE ,	
	bForceOpen_In		:= aForceOpValve[103],
	bValveInterlock_In	:= aILK_AV[103] ,		
	bPMCCtrl_In			:= GVL.stPMCtoPLC.aAV[103] ,
	bValveOpen_Out		=> aAV[103] 	
);				
				
AV[104]				
(	bValveEnable_In 	:= TRUE ,		
	bInterlock1_In		:= bEMOStatus ,	
	bInterlock2_In		:= TRUE ,	
	bInterlock3_In		:= TRUE ,	
	bInterlock4_In		:= TRUE ,	
	bInterlock5_In		:= TRUE ,	
	bForceOpen_In		:= aForceOpValve[104],
	bValveInterlock_In	:= aILK_AV[104] ,		
	bPMCCtrl_In			:= GVL.stPMCtoPLC.aAV[104] ,
	bValveOpen_Out		=> aAV[104] 	
);				
				
AV[105]				
(	bValveEnable_In 	:= TRUE ,		
	bInterlock1_In		:= bEMOStatus ,	
	bInterlock2_In		:= TRUE ,	
	bInterlock3_In		:= TRUE ,	
	bInterlock4_In		:= TRUE ,	
	bInterlock5_In		:= TRUE ,	
	bForceOpen_In		:= aForceOpValve[105],
	bValveInterlock_In	:= aILK_AV[105] ,		
	bPMCCtrl_In			:= GVL.stPMCtoPLC.aAV[105] ,
	bValveOpen_Out		=> aAV[105] 	
);				
				
AV[106]				
(	bValveEnable_In 	:= TRUE ,		
	bInterlock1_In		:= bEMOStatus ,	
	bInterlock2_In		:= TRUE ,	
	bInterlock3_In		:= TRUE ,	
	bInterlock4_In		:= TRUE ,	
	bInterlock5_In		:= TRUE ,	
	bForceOpen_In		:= aForceOpValve[106],
	bValveInterlock_In	:= aILK_AV[106] ,		
	bPMCCtrl_In			:= GVL.stPMCtoPLC.aAV[106] ,
	bValveOpen_Out		=> aAV[106] 	
);				
				
AV[107]				
(	bValveEnable_In 	:= TRUE ,		
	bInterlock1_In		:= bEMOStatus ,	
	bInterlock2_In		:= TRUE ,	
	bInterlock3_In		:= TRUE ,	
	bInterlock4_In		:= TRUE ,	
	bInterlock5_In		:= TRUE ,	
	bForceOpen_In		:= aForceOpValve[107],
	bValveInterlock_In	:= aILK_AV[107] ,		
	bPMCCtrl_In			:= GVL.stPMCtoPLC.aAV[107] ,
	bValveOpen_Out		=> aAV[107] 	
);				
				
AV[108]				
(	bValveEnable_In 	:= TRUE ,		
	bInterlock1_In		:= bEMOStatus ,	
	bInterlock2_In		:= TRUE ,	
	bInterlock3_In		:= TRUE ,	
	bInterlock4_In		:= TRUE ,	
	bInterlock5_In		:= TRUE ,	
	bForceOpen_In		:= aForceOpValve[108],
	bValveInterlock_In	:= aILK_AV[108] ,		
	bPMCCtrl_In			:= GVL.stPMCtoPLC.aAV[108] ,
	bValveOpen_Out		=> aAV[108] 	
);				
				
AV[109]				
(	bValveEnable_In 	:= TRUE ,		
	bInterlock1_In		:= bEMOStatus ,	
	bInterlock2_In		:= TRUE ,	
	bInterlock3_In		:= TRUE ,	
	bInterlock4_In		:= TRUE ,	
	bInterlock5_In		:= TRUE ,	
	bForceOpen_In		:= aForceOpValve[109],
	bValveInterlock_In	:= aILK_AV[109] ,		
	bPMCCtrl_In			:= GVL.stPMCtoPLC.aAV[109] ,
	bValveOpen_Out		=> aAV[109] 	
);				
				
AV[110]				
(	bValveEnable_In 	:= TRUE ,		
	bInterlock1_In		:= bEMOStatus ,	
	bInterlock2_In		:= TRUE ,	
	bInterlock3_In		:= TRUE ,	
	bInterlock4_In		:= TRUE ,	
	bInterlock5_In		:= TRUE ,	
	bForceOpen_In		:= aForceOpValve[110],
	bValveInterlock_In	:= aILK_AV[110] ,		
	bPMCCtrl_In			:= GVL.stPMCtoPLC.aAV[110] ,
	bValveOpen_Out		=> aAV[110] 	
);				
				
AV[111]				
(	bValveEnable_In 	:= TRUE ,		
	bInterlock1_In		:= bEMOStatus ,	
	bInterlock2_In		:= TRUE ,	
	bInterlock3_In		:= TRUE ,	
	bInterlock4_In		:= TRUE ,	
	bInterlock5_In		:= TRUE ,
	bForceOpen_In		:= aForceOpValve[111],	
	bValveInterlock_In	:= aILK_AV[111] ,		
	bPMCCtrl_In			:= GVL.stPMCtoPLC.aAV[111] ,
	bValveOpen_Out		=> aAV[111] 	
);				
				
AV[112]				
(	bValveEnable_In 	:= TRUE ,		
	bInterlock1_In		:= bEMOStatus ,	
	bInterlock2_In		:= TRUE ,	
	bInterlock3_In		:= TRUE ,	
	bInterlock4_In		:= TRUE ,	
	bInterlock5_In		:= TRUE ,	
	bForceOpen_In		:= aForceOpValve[112],
	bValveInterlock_In	:= aILK_AV[112] ,		
	bPMCCtrl_In			:= GVL.stPMCtoPLC.aAV[112] ,
	bValveOpen_Out		=> aAV[112] 	
);				
				
AV[113]				
(	bValveEnable_In 	:= TRUE ,		
	bInterlock1_In		:= bEMOStatus ,	
	bInterlock2_In		:= TRUE ,	
	bInterlock3_In		:= TRUE ,	
	bInterlock4_In		:= TRUE ,	
	bInterlock5_In		:= TRUE ,	
	bForceOpen_In		:= aForceOpValve[113],
	bValveInterlock_In	:= aILK_AV[113] ,		
	bPMCCtrl_In			:= GVL.stPMCtoPLC.aAV[113] ,
	bValveOpen_Out		=> aAV[113] 	
);				
				
AV[114]				
(	bValveEnable_In 	:= TRUE ,		
	bInterlock1_In		:= bEMOStatus ,	
	bInterlock2_In		:= TRUE ,	
	bInterlock3_In		:= TRUE ,	
	bInterlock4_In		:= TRUE ,	
	bInterlock5_In		:= TRUE ,	
	bForceOpen_In		:= aForceOpValve[114],
	bValveInterlock_In	:= aILK_AV[114] ,		
	bPMCCtrl_In			:= GVL.stPMCtoPLC.aAV[114] ,
	bValveOpen_Out		=> aAV[114] 	
);				
				
AV[115]				
(	bValveEnable_In 	:= TRUE ,		
	bInterlock1_In		:= bEMOStatus ,	
	bInterlock2_In		:= TRUE ,	
	bInterlock3_In		:= TRUE ,	
	bInterlock4_In		:= TRUE ,	
	bInterlock5_In		:= TRUE ,	
	bForceOpen_In		:= aForceOpValve[115],
	bValveInterlock_In	:= aILK_AV[115] ,		
	bPMCCtrl_In			:= GVL.stPMCtoPLC.aAV[115] ,
	bValveOpen_Out		=> aAV[115] 	
);				
				
AV[116]				
(	bValveEnable_In 	:= TRUE ,		
	bInterlock1_In		:= bEMOStatus ,	
	bInterlock2_In		:= TRUE ,	
	bInterlock3_In		:= TRUE ,	
	bInterlock4_In		:= TRUE ,	
	bInterlock5_In		:= TRUE ,	
	bForceOpen_In		:= aForceOpValve[116],
	bValveInterlock_In	:= aILK_AV[116] ,		
	bPMCCtrl_In			:= GVL.stPMCtoPLC.aAV[116] ,
	bValveOpen_Out		=> aAV[116] 	
);				
				
AV[117]				
(	bValveEnable_In 	:= TRUE ,		
	bInterlock1_In		:= bEMOStatus ,	
	bInterlock2_In		:= TRUE ,	
	bInterlock3_In		:= TRUE ,	
	bInterlock4_In		:= TRUE ,	
	bInterlock5_In		:= TRUE ,	
	bForceOpen_In		:= aForceOpValve[117],
	bValveInterlock_In	:= aILK_AV[117] ,		
	bPMCCtrl_In			:= GVL.stPMCtoPLC.aAV[117] ,
	bValveOpen_Out		=> aAV[117] 	
);				
				
AV[118]				
(	bValveEnable_In 	:= TRUE ,		
	bInterlock1_In		:= bEMOStatus ,	
	bInterlock2_In		:= TRUE ,	
	bInterlock3_In		:= TRUE ,	
	bInterlock4_In		:= TRUE ,	
	bInterlock5_In		:= TRUE ,	
	bForceOpen_In		:= aForceOpValve[118],
	bValveInterlock_In	:= aILK_AV[118] ,		
	bPMCCtrl_In			:= GVL.stPMCtoPLC.aAV[118] ,
	bValveOpen_Out		=> aAV[118] 	
);				
				
AV[119]				
(	bValveEnable_In 	:= TRUE ,		
	bInterlock1_In		:= bEMOStatus ,	
	bInterlock2_In		:= TRUE ,	
	bInterlock3_In		:= TRUE ,	
	bInterlock4_In		:= TRUE ,	
	bInterlock5_In		:= TRUE ,	
	bForceOpen_In		:= aForceOpValve[119],
	bValveInterlock_In	:= aILK_AV[119] ,		
	bPMCCtrl_In			:= GVL.stPMCtoPLC.aAV[119] ,
	bValveOpen_Out		=> aAV[119] 	
);				
				
AV[120]				
(	bValveEnable_In 	:= TRUE ,		
	bInterlock1_In		:= bEMOStatus ,	
	bInterlock2_In		:= TRUE ,	
	bInterlock3_In		:= TRUE ,	
	bInterlock4_In		:= TRUE ,	
	bInterlock5_In		:= TRUE ,	
	bForceOpen_In		:= aForceOpValve[120],
	bValveInterlock_In	:= aILK_AV[120] ,		
	bPMCCtrl_In			:= GVL.stPMCtoPLC.aAV[120] ,
	bValveOpen_Out		=> aAV[120] 	
);				
				
AV[121]				
(	bValveEnable_In 	:= TRUE ,		
	bInterlock1_In		:= bEMOStatus ,	
	bInterlock2_In		:= TRUE ,	
	bInterlock3_In		:= TRUE ,	
	bInterlock4_In		:= TRUE ,	
	bInterlock5_In		:= TRUE ,	
	bForceOpen_In		:= aForceOpValve[121],
	bValveInterlock_In	:= aILK_AV[121] ,		
	bPMCCtrl_In			:= GVL.stPMCtoPLC.aAV[121] ,
	bValveOpen_Out		=> aAV[121] 	
);				
				
AV[122]				
(	bValveEnable_In 	:= TRUE ,		
	bInterlock1_In		:= bEMOStatus ,	
	bInterlock2_In		:= TRUE ,	
	bInterlock3_In		:= TRUE ,	
	bInterlock4_In		:= TRUE ,	
	bInterlock5_In		:= TRUE ,	
	bForceOpen_In		:= aForceOpValve[122],
	bValveInterlock_In	:= aILK_AV[122] ,		
	bPMCCtrl_In			:= GVL.stPMCtoPLC.aAV[122] ,
	bValveOpen_Out		=> aAV[122] 	
);				
				
AV[123]				
(	bValveEnable_In 	:= TRUE ,		
	bInterlock1_In		:= bEMOStatus ,	
	bInterlock2_In		:= TRUE ,	
	bInterlock3_In		:= TRUE ,	
	bInterlock4_In		:= TRUE ,	
	bInterlock5_In		:= TRUE ,	
	bForceOpen_In		:= aForceOpValve[123],
	bValveInterlock_In	:= aILK_AV[123] ,		
	bPMCCtrl_In			:= GVL.stPMCtoPLC.aAV[123] ,
	bValveOpen_Out		=> aAV[123] 	
);				
				
AV[124]				
(	bValveEnable_In 	:= TRUE ,		
	bInterlock1_In		:= bEMOStatus ,	
	bInterlock2_In		:= TRUE ,	
	bInterlock3_In		:= TRUE ,	
	bInterlock4_In		:= TRUE ,	
	bInterlock5_In		:= TRUE ,	
	bForceOpen_In		:= aForceOpValve[124],
	bValveInterlock_In	:= aILK_AV[124] ,		
	bPMCCtrl_In			:= GVL.stPMCtoPLC.aAV[124] ,
	bValveOpen_Out		=> aAV[124] 	
);				
				
AV[125]				
(	bValveEnable_In 	:= TRUE ,		
	bInterlock1_In		:= bEMOStatus ,	
	bInterlock2_In		:= TRUE ,	
	bInterlock3_In		:= TRUE ,	
	bInterlock4_In		:= TRUE ,	
	bInterlock5_In		:= TRUE ,	
	bForceOpen_In		:= aForceOpValve[125],
	bValveInterlock_In	:= aILK_AV[125] ,		
	bPMCCtrl_In			:= GVL.stPMCtoPLC.aAV[125] ,
	bValveOpen_Out		=> aAV[125] 	
);				
				
AV[126]				
(	bValveEnable_In 	:= TRUE ,		
	bInterlock1_In		:= bEMOStatus ,	
	bInterlock2_In		:= TRUE ,	
	bInterlock3_In		:= TRUE ,	
	bInterlock4_In		:= TRUE ,	
	bInterlock5_In		:= TRUE ,	
	bForceOpen_In		:= aForceOpValve[126],
	bValveInterlock_In	:= aILK_AV[126] ,		
	bPMCCtrl_In			:= GVL.stPMCtoPLC.aAV[126] ,
	bValveOpen_Out		=> aAV[126] 	
);				
				
AV[127]				
(	bValveEnable_In 	:= TRUE ,		
	bInterlock1_In		:= bEMOStatus ,	
	bInterlock2_In		:= TRUE ,	
	bInterlock3_In		:= TRUE ,	
	bInterlock4_In		:= TRUE ,	
	bInterlock5_In		:= TRUE ,	
	bForceOpen_In		:= aForceOpValve[127],
	bValveInterlock_In	:= aILK_AV[127] ,		
	bPMCCtrl_In			:= GVL.stPMCtoPLC.aAV[127] ,
	bValveOpen_Out		=> aAV[127] 	
);				
				
AV[128]				
(	bValveEnable_In 	:= TRUE ,		
	bInterlock1_In		:= bEMOStatus ,	
	bInterlock2_In		:= TRUE ,	
	bInterlock3_In		:= TRUE ,	
	bInterlock4_In		:= TRUE ,	
	bInterlock5_In		:= TRUE ,	
	bForceOpen_In		:= aForceOpValve[128],
	bValveInterlock_In	:= aILK_AV[128] ,		
	bPMCCtrl_In			:= GVL.stPMCtoPLC.aAV[128] ,
	bValveOpen_Out		=> aAV[128] 	
);				
				
AV[129]				
(	bValveEnable_In 	:= TRUE ,		
	bInterlock1_In		:= bEMOStatus ,	
	bInterlock2_In		:= TRUE ,	
	bInterlock3_In		:= TRUE ,	
	bInterlock4_In		:= TRUE ,	
	bInterlock5_In		:= TRUE ,	
	bForceOpen_In		:= aForceOpValve[129],
	bValveInterlock_In	:= aILK_AV[129] ,		
	bPMCCtrl_In			:= GVL.stPMCtoPLC.aAV[129] ,
	bValveOpen_Out		=> aAV[129] 	
);				
				
AV[130]				
(	bValveEnable_In 	:= TRUE ,		
	bInterlock1_In		:= bEMOStatus ,	
	bInterlock2_In		:= TRUE ,	
	bInterlock3_In		:= TRUE ,	
	bInterlock4_In		:= TRUE ,	
	bInterlock5_In		:= TRUE ,	
	bForceOpen_In		:= aForceOpValve[130],
	bValveInterlock_In	:= aILK_AV[130] ,		
	bPMCCtrl_In			:= GVL.stPMCtoPLC.aAV[130] ,
	bValveOpen_Out		=> aAV[130] 	
);				
				
AV[131]				
(	bValveEnable_In 	:= TRUE ,		
	bInterlock1_In		:= bEMOStatus ,	
	bInterlock2_In		:= TRUE ,	
	bInterlock3_In		:= TRUE ,	
	bInterlock4_In		:= TRUE ,	
	bInterlock5_In		:= TRUE ,	
	bForceOpen_In		:= aForceOpValve[131],
	bValveInterlock_In	:= aILK_AV[131] ,		
	bPMCCtrl_In			:= GVL.stPMCtoPLC.aAV[131] ,
	bValveOpen_Out		=> aAV[131] 	
);				
				
AV[132]				
(	bValveEnable_In 	:= TRUE ,		
	bInterlock1_In		:= bEMOStatus ,	
	bInterlock2_In		:= TRUE ,	
	bInterlock3_In		:= TRUE ,	
	bInterlock4_In		:= TRUE ,	
	bInterlock5_In		:= TRUE ,	
	bForceOpen_In		:= aForceOpValve[132],
	bValveInterlock_In	:= aILK_AV[132] ,		
	bPMCCtrl_In			:= GVL.stPMCtoPLC.aAV[132] ,
	bValveOpen_Out		=> aAV[132] 	
);				
				
AV[133]				
(	bValveEnable_In 	:= TRUE ,		
	bInterlock1_In		:= bEMOStatus ,	
	bInterlock2_In		:= TRUE ,	
	bInterlock3_In		:= TRUE ,	
	bInterlock4_In		:= TRUE ,	
	bInterlock5_In		:= TRUE ,	
	bForceOpen_In		:= aForceOpValve[133],
	bValveInterlock_In	:= aILK_AV[133] ,		
	bPMCCtrl_In			:= GVL.stPMCtoPLC.aAV[133] ,
	bValveOpen_Out		=> aAV[133] 	
);				
				
AV[134]				
(	bValveEnable_In 	:= TRUE ,		
	bInterlock1_In		:= bEMOStatus ,	
	bInterlock2_In		:= TRUE ,	
	bInterlock3_In		:= TRUE ,	
	bInterlock4_In		:= TRUE ,	
	bInterlock5_In		:= TRUE ,	
	bForceOpen_In		:= aForceOpValve[134],
	bValveInterlock_In	:= aILK_AV[134] ,		
	bPMCCtrl_In			:= GVL.stPMCtoPLC.aAV[134] ,
	bValveOpen_Out		=> aAV[134] 	
);				
				
AV[135]				
(	bValveEnable_In 	:= TRUE ,		
	bInterlock1_In		:= bEMOStatus ,	
	bInterlock2_In		:= TRUE ,	
	bInterlock3_In		:= TRUE ,	
	bInterlock4_In		:= TRUE ,	
	bInterlock5_In		:= TRUE ,	
	bForceOpen_In		:= aForceOpValve[135],
	bValveInterlock_In	:= aILK_AV[135] ,		
	bPMCCtrl_In			:= GVL.stPMCtoPLC.aAV[135] ,
	bValveOpen_Out		=> aAV[135] 	
);				
				
AV[136]				
(	bValveEnable_In 	:= TRUE ,		
	bInterlock1_In		:= bEMOStatus ,	
	bInterlock2_In		:= TRUE ,	
	bInterlock3_In		:= TRUE ,	
	bInterlock4_In		:= TRUE ,	
	bInterlock5_In		:= TRUE ,	
	bForceOpen_In		:= aForceOpValve[136],
	bValveInterlock_In	:= aILK_AV[136] ,		
	bPMCCtrl_In			:= GVL.stPMCtoPLC.aAV[136] ,
	bValveOpen_Out		=> aAV[136] 	
);				
				
AV[137]				
(	bValveEnable_In 	:= TRUE ,		
	bInterlock1_In		:= bEMOStatus ,	
	bInterlock2_In		:= TRUE ,	
	bInterlock3_In		:= TRUE ,	
	bInterlock4_In		:= TRUE ,	
	bInterlock5_In		:= TRUE ,	
	bForceOpen_In		:= aForceOpValve[137],
	bValveInterlock_In	:= aILK_AV[137] ,		
	bPMCCtrl_In			:= GVL.stPMCtoPLC.aAV[137] ,
	bValveOpen_Out		=> aAV[137] 	
);				
				
AV[138]				
(	bValveEnable_In 	:= TRUE ,		
	bInterlock1_In		:= bEMOStatus ,	
	bInterlock2_In		:= TRUE ,	
	bInterlock3_In		:= TRUE ,	
	bInterlock4_In		:= TRUE ,	
	bInterlock5_In		:= TRUE ,	
	bForceOpen_In		:= aForceOpValve[138],
	bValveInterlock_In	:= aILK_AV[138] ,		
	bPMCCtrl_In			:= GVL.stPMCtoPLC.aAV[138] ,
	bValveOpen_Out		=> aAV[138] 	
);				
				
AV[139]				
(	bValveEnable_In 	:= TRUE ,		
	bInterlock1_In		:= bEMOStatus ,	
	bInterlock2_In		:= TRUE ,	
	bInterlock3_In		:= TRUE ,	
	bInterlock4_In		:= TRUE ,	
	bInterlock5_In		:= TRUE ,	
	bForceOpen_In		:= aForceOpValve[139],
	bValveInterlock_In	:= aILK_AV[139] ,		
	bPMCCtrl_In			:= GVL.stPMCtoPLC.aAV[139] ,
	bValveOpen_Out		=> aAV[139] 	
);				
				
AV[140]				
(	bValveEnable_In 	:= TRUE ,		
	bInterlock1_In		:= bEMOStatus ,	
	bInterlock2_In		:= TRUE ,	
	bInterlock3_In		:= TRUE ,	
	bInterlock4_In		:= TRUE ,	
	bInterlock5_In		:= TRUE ,	
	bForceOpen_In		:= aForceOpValve[140],
	bValveInterlock_In	:= aILK_AV[140] ,		
	bPMCCtrl_In			:= GVL.stPMCtoPLC.aAV[140] ,
	bValveOpen_Out		=> aAV[140] 	
);				
				
AV[141]				
(	bValveEnable_In 	:= TRUE ,		
	bInterlock1_In		:= bEMOStatus ,	
	bInterlock2_In		:= TRUE ,	
	bInterlock3_In		:= TRUE ,	
	bInterlock4_In		:= TRUE ,	
	bInterlock5_In		:= TRUE ,	
	bForceOpen_In		:= aForceOpValve[141],
	bValveInterlock_In	:= aILK_AV[141] ,		
	bPMCCtrl_In			:= GVL.stPMCtoPLC.aAV[141] ,
	bValveOpen_Out		=> aAV[141] 	
);				
				
AV[142]				
(	bValveEnable_In 	:= TRUE ,		
	bInterlock1_In		:= bEMOStatus ,	
	bInterlock2_In		:= TRUE ,	
	bInterlock3_In		:= TRUE ,	
	bInterlock4_In		:= TRUE ,	
	bInterlock5_In		:= TRUE ,	
	bForceOpen_In		:= aForceOpValve[142],
	bValveInterlock_In	:= aILK_AV[142] ,		
	bPMCCtrl_In			:= GVL.stPMCtoPLC.aAV[142] ,
	bValveOpen_Out		=> aAV[142] 	
);				
				
AV[143]				
(	bValveEnable_In 	:= TRUE ,		
	bInterlock1_In		:= bEMOStatus ,	
	bInterlock2_In		:= TRUE ,	
	bInterlock3_In		:= TRUE ,	
	bInterlock4_In		:= TRUE ,	
	bInterlock5_In		:= TRUE ,	
	bForceOpen_In		:= aForceOpValve[143],
	bValveInterlock_In	:= aILK_AV[143] ,		
	bPMCCtrl_In			:= GVL.stPMCtoPLC.aAV[143] ,
	bValveOpen_Out		=> aAV[143] 	
);				
				
AV[144]				
(	bValveEnable_In 	:= TRUE ,		
	bInterlock1_In		:= bEMOStatus ,	
	bInterlock2_In		:= TRUE ,	
	bInterlock3_In		:= TRUE ,	
	bInterlock4_In		:= TRUE ,	
	bInterlock5_In		:= TRUE ,	
	bForceOpen_In		:= aForceOpValve[144],
	bValveInterlock_In	:= aILK_AV[144] ,		
	bPMCCtrl_In			:= GVL.stPMCtoPLC.aAV[144] ,
	bValveOpen_Out		=> aAV[144] 	
);				
				
AV[145]				
(	bValveEnable_In 	:= TRUE ,		
	bInterlock1_In		:= bEMOStatus ,	
	bInterlock2_In		:= TRUE ,	
	bInterlock3_In		:= TRUE ,	
	bInterlock4_In		:= TRUE ,	
	bInterlock5_In		:= TRUE ,	
	bForceOpen_In		:= aForceOpValve[145],
	bValveInterlock_In	:= aILK_AV[145] ,		
	bPMCCtrl_In			:= GVL.stPMCtoPLC.aAV[145] ,
	bValveOpen_Out		=> aAV[145] 	
);				
				
AV[146]				
(	bValveEnable_In 	:= TRUE ,		
	bInterlock1_In		:= bEMOStatus ,	
	bInterlock2_In		:= TRUE ,	
	bInterlock3_In		:= TRUE ,	
	bInterlock4_In		:= TRUE ,	
	bInterlock5_In		:= TRUE ,	
	bForceOpen_In		:= aForceOpValve[146],
	bValveInterlock_In	:= aILK_AV[146] ,		
	bPMCCtrl_In			:= GVL.stPMCtoPLC.aAV[146] ,
	bValveOpen_Out		=> aAV[146] 	
);				
				
AV[147]				
(	bValveEnable_In 	:= TRUE ,		
	bInterlock1_In		:= bEMOStatus ,	
	bInterlock2_In		:= TRUE ,	
	bInterlock3_In		:= TRUE ,	
	bInterlock4_In		:= TRUE ,	
	bInterlock5_In		:= TRUE ,	
	bForceOpen_In		:= aForceOpValve[147],
	bValveInterlock_In	:= aILK_AV[147] ,		
	bPMCCtrl_In			:= GVL.stPMCtoPLC.aAV[147] ,
	bValveOpen_Out		=> aAV[147] 	
);				
				
AV[148]				
(	bValveEnable_In 	:= TRUE ,		
	bInterlock1_In		:= bEMOStatus ,	
	bInterlock2_In		:= TRUE ,	
	bInterlock3_In		:= TRUE ,	
	bInterlock4_In		:= TRUE ,	
	bInterlock5_In		:= TRUE ,	
	bForceOpen_In		:= aForceOpValve[148],
	bValveInterlock_In	:= aILK_AV[148] ,		
	bPMCCtrl_In			:= GVL.stPMCtoPLC.aAV[148] ,
	bValveOpen_Out		=> aAV[148] 	
);				
				
AV[149]				
(	bValveEnable_In 	:= TRUE ,		
	bInterlock1_In		:= bEMOStatus ,	
	bInterlock2_In		:= TRUE ,	
	bInterlock3_In		:= TRUE ,	
	bInterlock4_In		:= TRUE ,	
	bInterlock5_In		:= TRUE ,	
	bForceOpen_In		:= aForceOpValve[149],
	bValveInterlock_In	:= aILK_AV[149] ,		
	bPMCCtrl_In			:= GVL.stPMCtoPLC.aAV[149] ,
	bValveOpen_Out		=> aAV[149] 	
);				
				
AV[150]				
(	bValveEnable_In 	:= TRUE ,		
	bInterlock1_In		:= bEMOStatus ,	
	bInterlock2_In		:= TRUE ,	
	bInterlock3_In		:= TRUE ,	
	bInterlock4_In		:= TRUE ,	
	bInterlock5_In		:= TRUE ,	
	bForceOpen_In		:= aForceOpValve[150],
	bValveInterlock_In	:= aILK_AV[150] ,		
	bPMCCtrl_In			:= GVL.stPMCtoPLC.aAV[150] ,
	bValveOpen_Out		=> aAV[150] 	
);		

(*AV[202]
(	bValveEnable_In 	:= TRUE ,		
	bInterlock1_In		:= bEMOStatus ,	
	bInterlock2_In		:= TRUE ,	
	bInterlock3_In		:= TRUE ,	
	bInterlock4_In		:= TRUE ,	
	bInterlock5_In		:= TRUE ,	
	bForceOpen_In		:= aForceOpValve[150],
	bValveInterlock_In	:= TRUE(*aILK_AV[202]*) ,		
	bPMCCtrl_In			:= GVL.stPMCtoPLC.aAV[202] ,
	bValveOpen_Out		=> aAV[202] 	
);	*)

AV202Open				
(	bValveEnable_In 	:= TRUE ,		
	bInterlock1_In		:= bEMOStatus ,	
	bInterlock2_In		:= TRUE ,	
	bInterlock3_In		:= TRUE ,	
	bInterlock4_In		:= TRUE ,	
	bInterlock5_In		:= TRUE ,
	bForceOpen_In		:= bForceAV202Open,	
	bValveInterlock_In	:= aILK_AV[202] ,		
	bPMCCtrl_In			:= GVL.stPMCtoPLC.bAV202Open ,
	bValveOpen_Out		=> GVL.bAV202Open 	
);	

AV202Close				
(	bValveEnable_In 	:= TRUE ,		
	bInterlock1_In		:= bEMOStatus ,	
	bInterlock2_In		:= TRUE ,	
	bInterlock3_In		:= TRUE ,	
	bInterlock4_In		:= TRUE ,	
	bInterlock5_In		:= TRUE ,
	bForceOpen_In		:= bForceAV202Close,	
	bValveInterlock_In	:= aILK_AV[202] ,		
	bPMCCtrl_In			:= GVL.stPMCtoPLC.bAV202Close ,
	bValveOpen_Out		=> GVL.bAV202Close 	
);
END_ACTION

ACTION ValveMapping:
//interlock mapping
GVL.stPLCtoPMC.stIntlk := stILK ; 

//valve interlock mapping
GVL.stPLCtoPMC.aILK_AV := aILK_AV ;

//VAC mapping
GVL.stPLCtoPMC.aVAC		:= aVAC ;

//AV540
GVL.stPLCtoPMC.bAV540	:= bAV540 ;

(*EV1*)
//stGBQ.QEV[1].A.uBit.v1	:=  aAV[];
stGBQ.QEV[1].A.uBit.v2	:=  aAV[52];
//stGBQ.QEV[1].A.uBit.v3	:=  aAV[];
stGBQ.QEV[1].A.uBit.v4	:=  aAV[100];
//stGBQ.QEV[1].A.uBit.v5	:=  aAV[];
stGBQ.QEV[1].A.uBit.v6	:=  aAV[102];
stGBQ.QEV[1].A.uBit.v7	:=  aAV[103];
stGBQ.QEV[1].A.uBit.v8	:=  aAV[104];
	
stGBQ.QEV[1].B.uBit.v1	:=  aAV[105];
stGBQ.QEV[1].B.uBit.v2	:=  aAV[106];
stGBQ.QEV[1].B.uBit.v3	:=  aAV[107];
//stGBQ.QEV[1].B.uBit.v4	:=  aAV[];
//stGBQ.QEV[1].B.uBit.v5	:=  aAV[];
stGBQ.QEV[1].B.uBit.v6	:=  aAV[110];
//stGBQ.QEV[1].B.uBit.v7	:=  aAV[];
stGBQ.QEV[1].B.uBit.v8	:=  aAV[112];
	
//stGBQ.QEV[1].C.uBit.v1	:=  aAV[];
stGBQ.QEV[1].C.uBit.v2	:=  aAV[120];
stGBQ.QEV[1].C.uBit.v3	:=  aAV[121];
stGBQ.QEV[1].C.uBit.v4	:=  aAV[122];
stGBQ.QEV[1].C.uBit.v5	:=  aAV[123];
stGBQ.QEV[1].C.uBit.v6	:=  aAV[124];
stGBQ.QEV[1].C.uBit.v7	:=  aAV[125];
stGBQ.QEV[1].C.uBit.v8	:=  aAV[126];
	
stGBQ.QEV[1].D.uBit.v1	:=  aAV[127];
stGBQ.QEV[1].D.uBit.v2	:=  aAV[128];
stGBQ.QEV[1].D.uBit.v3	:=  aAV[129];
stGBQ.QEV[1].D.uBit.v4	:=  aAV[130];
stGBQ.QEV[1].D.uBit.v5	:=  aAV[131];
//stGBQ.QEV[1].D.uBit.v6	:=  aAV[];
stGBQ.QEV[1].D.uBit.v7	:=  aAV[136];
stGBQ.QEV[1].D.uBit.v8	:=  aAV[137];


//EV2
stGBQ.QEV[2].A.uBit.v1	:=  aAV[101];
stGBQ.QEV[2].A.uBit.v2	:=  aAV[111];
//stGBQ.QEV[2].A.uBit.v3	:=  
//stGBQ.QEV[2].A.uBit.v4	:=  
//stGBQ.QEV[2].A.uBit.v5	:=  
//stGBQ.QEV[2].A.uBit.v6	:=  
//stGBQ.QEV[2].A.uBit.v7	:=  
//stGBQ.QEV[2].A.uBit.v8	:=  
	
(*sstGBQ.QEV[2].B.uBit.v1	:=  
stGBQ.QEV[2].B.uBit.v2	:=  
stGBQ.QEV[2].B.uBit.v3	:=  
stGBQ.QEV[2].B.uBit.v4	:=  
stGBQ.QEV[2].B.uBit.v5	:=  
stGBQ.QEV[2].B.uBit.v6	:=  
stGBQ.QEV[2].B.uBit.v7	:=  
stGBQ.QEV[2].B.uBit.v8	:=  
	
tGBQ.QEV[2].C.uBit.v1	:=  
stGBQ.QEV[2].C.uBit.v2	:=  
stGBQ.QEV[2].C.uBit.v3	:=  
stGBQ.QEV[2].C.uBit.v4	:=  
stGBQ.QEV[2].C.uBit.v5	:=  
stGBQ.QEV[2].C.uBit.v6	:=  
stGBQ.QEV[2].C.uBit.v7	:=  
stGBQ.QEV[2].C.uBit.v8	:=  
	
stGBQ.QEV[2].D.uBit.v1	:=  
stGBQ.QEV[2].D.uBit.v2	:=  
stGBQ.QEV[2].D.uBit.v3	:=  
stGBQ.QEV[2].D.uBit.v4	:=  
stGBQ.QEV[2].D.uBit.v5	:=  
stGBQ.QEV[2].D.uBit.v6	:=  
stGBQ.QEV[2].D.uBit.v7	:=  
stGBQ.QEV[2].D.uBit.v8	:=  *)

//EV3
stGBQ.QEV[3].A.uBit.v1	:=  aAV[1];
//stGBQ.QEV[3].A.uBit.v2	:=  aAV[];
stGBQ.QEV[3].A.uBit.v3	:=  aAV[3];
stGBQ.QEV[3].A.uBit.v4	:=  aAV[4];
stGBQ.QEV[3].A.uBit.v5	:=  aAV[5];
stGBQ.QEV[3].A.uBit.v6	:=  aAV[6];
stGBQ.QEV[3].A.uBit.v7	:=  aAV[7];
stGBQ.QEV[3].A.uBit.v8	:=  aAV[8];
	
stGBQ.QEV[3].B.uBit.v1	:=  aAV[9];
stGBQ.QEV[3].B.uBit.v2	:=  aAV[10];
stGBQ.QEV[3].B.uBit.v3	:=  aAV[11];
stGBQ.QEV[3].B.uBit.v4	:=  aAV[33];
stGBQ.QEV[3].B.uBit.v5	:=  aAV[13];
stGBQ.QEV[3].B.uBit.v6	:=  aAV[14];
stGBQ.QEV[3].B.uBit.v7	:=  aAV[15];
stGBQ.QEV[3].B.uBit.v8	:=  aAV[35];
	
stGBQ.QEV[3].C.uBit.v1	:=  aAV[17];
stGBQ.QEV[3].C.uBit.v2	:=  aAV[18];
stGBQ.QEV[3].C.uBit.v3	:=  aAV[19];
stGBQ.QEV[3].C.uBit.v4	:=  aAV[36];
stGBQ.QEV[3].C.uBit.v5	:=  aAV[21];
stGBQ.QEV[3].C.uBit.v6	:=  aAV[22];
stGBQ.QEV[3].C.uBit.v7	:=  aAV[23];
stGBQ.QEV[3].C.uBit.v8	:=  aAV[24];
	
stGBQ.QEV[3].D.uBit.v1	:=  aAV[25];
//stGBQ.QEV[3].D.uBit.v2	:=  aAV[];
stGBQ.QEV[3].D.uBit.v3	:=  aAV[27];
stGBQ.QEV[3].D.uBit.v4	:=  aAV[28];
stGBQ.QEV[3].D.uBit.v5	:=  aAV[29];
//stGBQ.QEV[3].D.uBit.v6	:=  aAV[];
stGBQ.QEV[3].D.uBit.v7	:=  aAV[31];
stGBQ.QEV[3].D.uBit.v8	:=  aAV[32];

//EV4
stGBQ.QEV[4].A.uBit.v1	:=  aAV[16];
stGBQ.QEV[4].A.uBit.v2	:=  aAV[12];
stGBQ.QEV[4].A.uBit.v3	:=  aAV[26];
stGBQ.QEV[4].A.uBit.v4	:=  aAV[20];
stGBQ.QEV[4].A.uBit.v5	:=  aAV[34];
stGBQ.QEV[4].A.uBit.v6	:=  aAV[30];
//stGBQ.QEV[4].A.uBit.v7	:=  aAV[];
//stGBQ.QEV[4].A.uBit.v8	:=  aAV[];
	
(*stGBQ.QEV[4].B.uBit.v1	:=  
stGBQ.QEV[4].B.uBit.v2	:=  
stGBQ.QEV[4].B.uBit.v3	:=  
stGBQ.QEV[4].B.uBit.v4	:=  
stGBQ.QEV[4].B.uBit.v5	:=  
stGBQ.QEV[4].B.uBit.v6	:=  
stGBQ.QEV[4].B.uBit.v7	:=  
stGBQ.QEV[4].B.uBit.v8	:=  
	
stGBQ.QEV[4].C.uBit.v1	:=  
stGBQ.QEV[4].C.uBit.v2	:=  
stGBQ.QEV[4].C.uBit.v3	:=  
stGBQ.QEV[4].C.uBit.v4	:=  
stGBQ.QEV[4].C.uBit.v5	:=  
stGBQ.QEV[4].C.uBit.v6	:=  
stGBQ.QEV[4].C.uBit.v7	:=  
stGBQ.QEV[4].C.uBit.v8	:=  
	
stGBQ.QEV[4].D.uBit.v1	:=  
stGBQ.QEV[4].D.uBit.v2	:=  
stGBQ.QEV[4].D.uBit.v3	:=  
stGBQ.QEV[4].D.uBit.v4	:=  
stGBQ.QEV[4].D.uBit.v5	:=  
stGBQ.QEV[4].D.uBit.v6	:=  
stGBQ.QEV[4].D.uBit.v7	:=  
stGBQ.QEV[4].D.uBit.v8	:=  *)

//EV5
stGBQ.QEV[5].A.uBit.v1	:=  GVL.bAV65Open;
stGBQ.QEV[5].A.uBit.v2	:=  GVL.bAV65Close;
stGBQ.QEV[5].A.uBit.v3	:=  GVL.bAV202Open;
stGBQ.QEV[5].A.uBit.v4	:=  GVL.bAV202Close;
//stGBQ.QEV[5].A.uBit.v5	:=  
//stGBQ.QEV[5].A.uBit.v6	:=  
//stGBQ.QEV[5].A.uBit.v7	:=  
//stGBQ.QEV[5].A.uBit.v8	:=  
	
(*stGBQ.QEV[5].B.uBit.v1	:=  
stGBQ.QEV[5].B.uBit.v2	:=  
stGBQ.QEV[5].B.uBit.v3	:=  
stGBQ.QEV[5].B.uBit.v4	:=  
stGBQ.QEV[5].B.uBit.v5	:=  
stGBQ.QEV[5].B.uBit.v6	:=  
stGBQ.QEV[5].B.uBit.v7	:=  
stGBQ.QEV[5].B.uBit.v8	:=  
	
stGBQ.QEV[5].C.uBit.v1	:=  
stGBQ.QEV[5].C.uBit.v2	:=  
stGBQ.QEV[5].C.uBit.v3	:=  
stGBQ.QEV[5].C.uBit.v4	:=  
stGBQ.QEV[5].C.uBit.v5	:=  
stGBQ.QEV[5].C.uBit.v6	:=  
stGBQ.QEV[5].C.uBit.v7	:=  
stGBQ.QEV[5].C.uBit.v8	:=  
	
stGBQ.QEV[5].D.uBit.v1	:=  
stGBQ.QEV[5].D.uBit.v2	:=  
stGBQ.QEV[5].D.uBit.v3	:=  
stGBQ.QEV[5].D.uBit.v4	:=  
stGBQ.QEV[5].D.uBit.v5	:=  
stGBQ.QEV[5].D.uBit.v6	:=  
stGBQ.QEV[5].D.uBit.v7	:=  
stGBQ.QEV[5].D.uBit.v8	:=  *)

//VT301
stEXHQ.QEV[1].A.uBit.v1	:=  GVL.bAV79Open(*aAV[78]*);
stEXHQ.QEV[1].A.uBit.v2	:=  GVL.bAV79Close(*aAV[78]*);
//stEXHQ.QEV[1].A.uBit.v3	:=  aAV[];
//stEXHQ.QEV[1].A.uBit.v4	:=  aAV[];
//stEXHQ.QEV[1].A.uBit.v5	:=  aAV[];
//stEXHQ.QEV[1].A.uBit.v6	:=  aAV[];
//stEXHQ.QEV[1].A.uBit.v7	:=  aAV[];
//stEXHQ.QEV[1].A.uBit.v8	:=  aAV[];
	
//stEXHQ.QEV[1].B.uBit.v1	:=  aAV[];
//stEXHQ.QEV[1].B.uBit.v2	:=  aAV[];
stEXHQ.QEV[1].B.uBit.v3	:=  GVL.bAV91Open;
stEXHQ.QEV[1].B.uBit.v4	:=  GVL.bAV91Close;
stEXHQ.QEV[1].B.uBit.v5	:=  FALSE(*aAV[71]*);
//stEXHQ.QEV[1].B.uBit.v6	:=  aAV[];
stEXHQ.QEV[1].B.uBit.v7	:=  aAV[60];
stEXHQ.QEV[1].B.uBit.v8	:=  aAV[67];
	
stEXHQ.QEV[1].C.uBit.v1	:=  aAV[68];
stEXHQ.QEV[1].C.uBit.v2	:=  aAV[72];
stEXHQ.QEV[1].C.uBit.v3	:=  aAV[73];
stEXHQ.QEV[1].C.uBit.v4	:=  aAV[74];
stEXHQ.QEV[1].C.uBit.v5	:=  aAV[75];
stEXHQ.QEV[1].C.uBit.v6	:=  aAV[77];
stEXHQ.QEV[1].C.uBit.v7	:=  aAV[85];
stEXHQ.QEV[1].C.uBit.v8	:=  aAV[86];
	
stEXHQ.QEV[1].D.uBit.v1	:=  aAV[87];
stEXHQ.QEV[1].D.uBit.v2	:=  aAV[88];
(*stEXHQ.QEV[1].D.uBit.v3	:=  
stEXHQ.QEV[1].D.uBit.v4	:=  
stEXHQ.QEV[1].D.uBit.v5	:=  
stEXHQ.QEV[1].D.uBit.v6	:=  
stEXHQ.QEV[1].D.uBit.v7	:=  
stEXHQ.QEV[1].D.uBit.v8	:=  *)
END_ACTION

END_PROGRAM
